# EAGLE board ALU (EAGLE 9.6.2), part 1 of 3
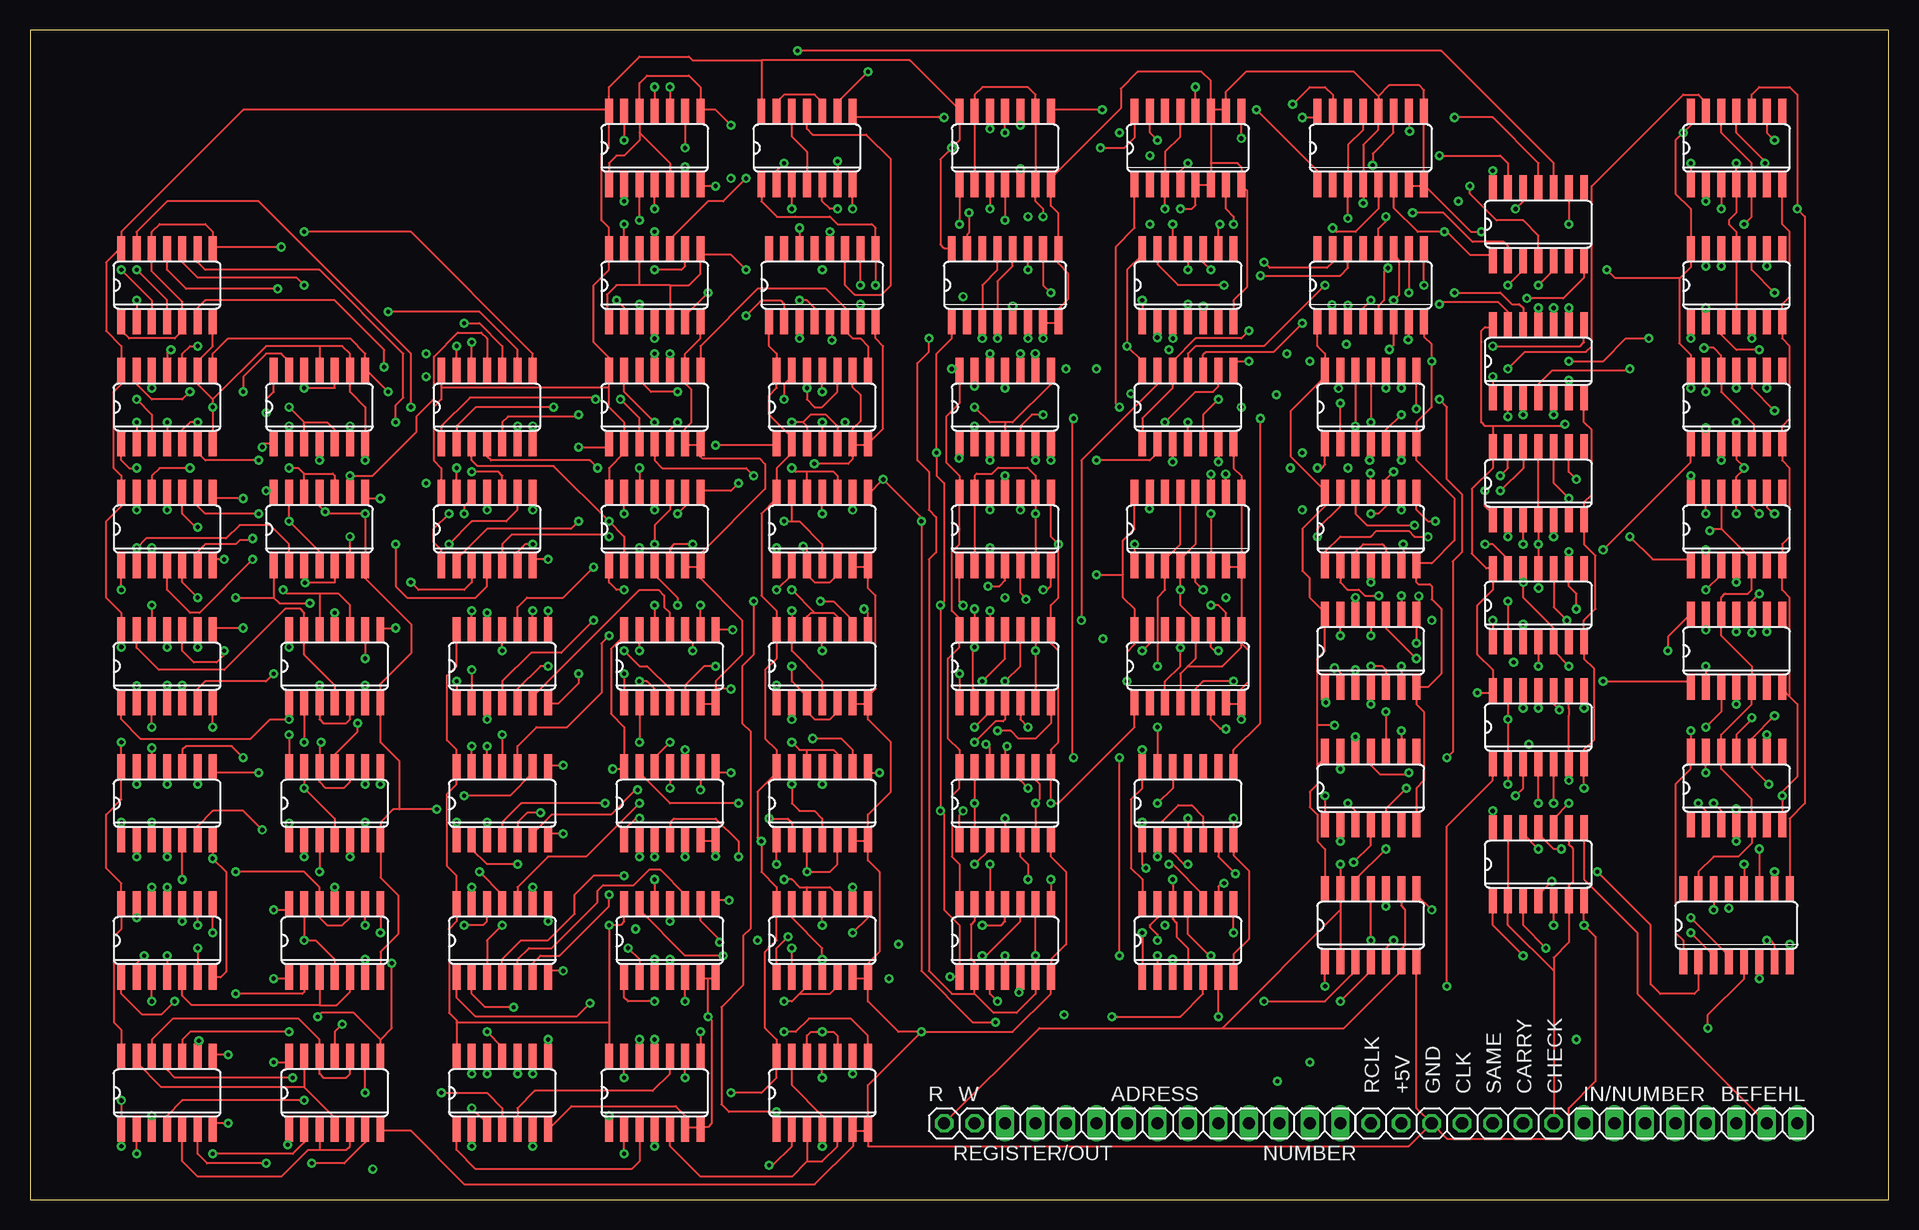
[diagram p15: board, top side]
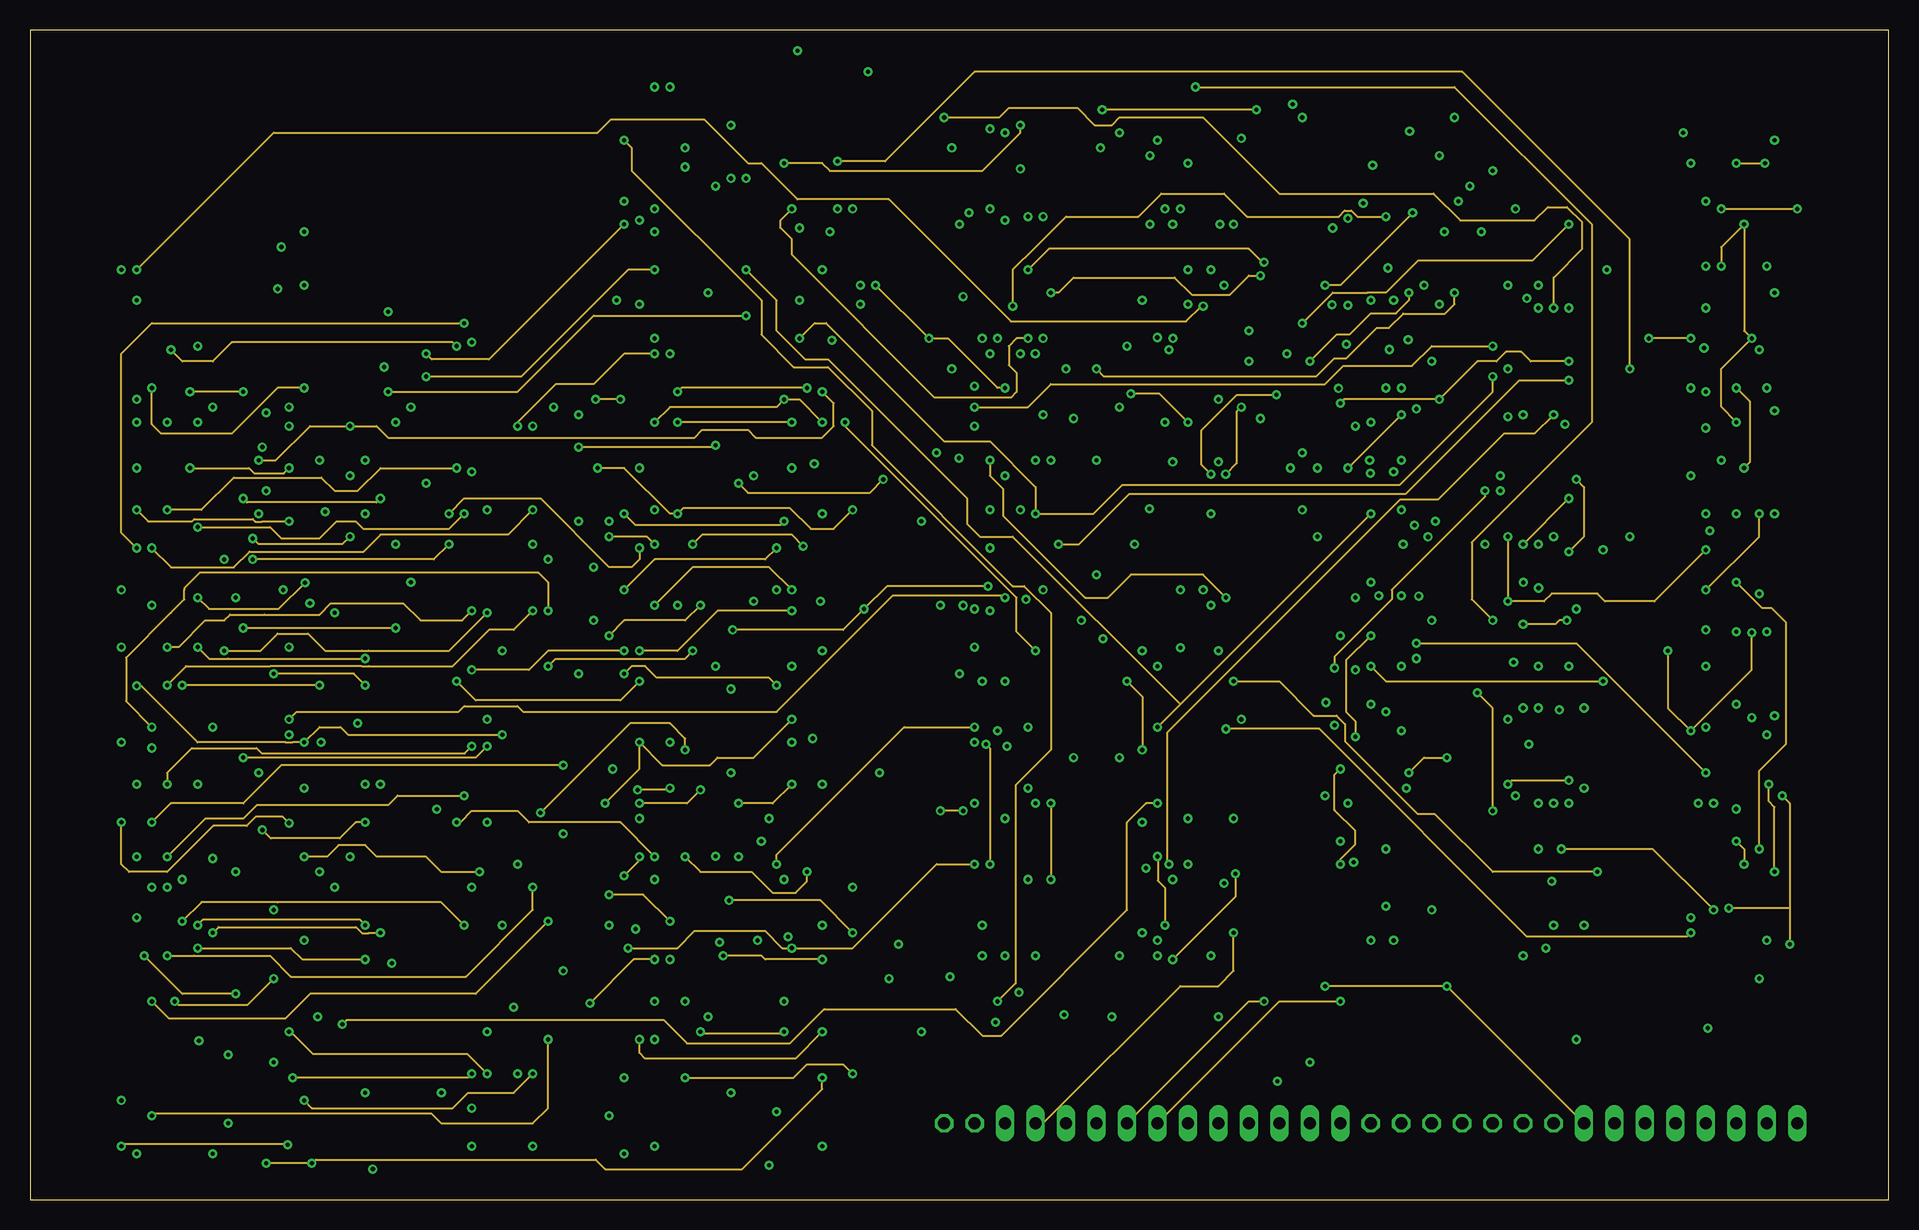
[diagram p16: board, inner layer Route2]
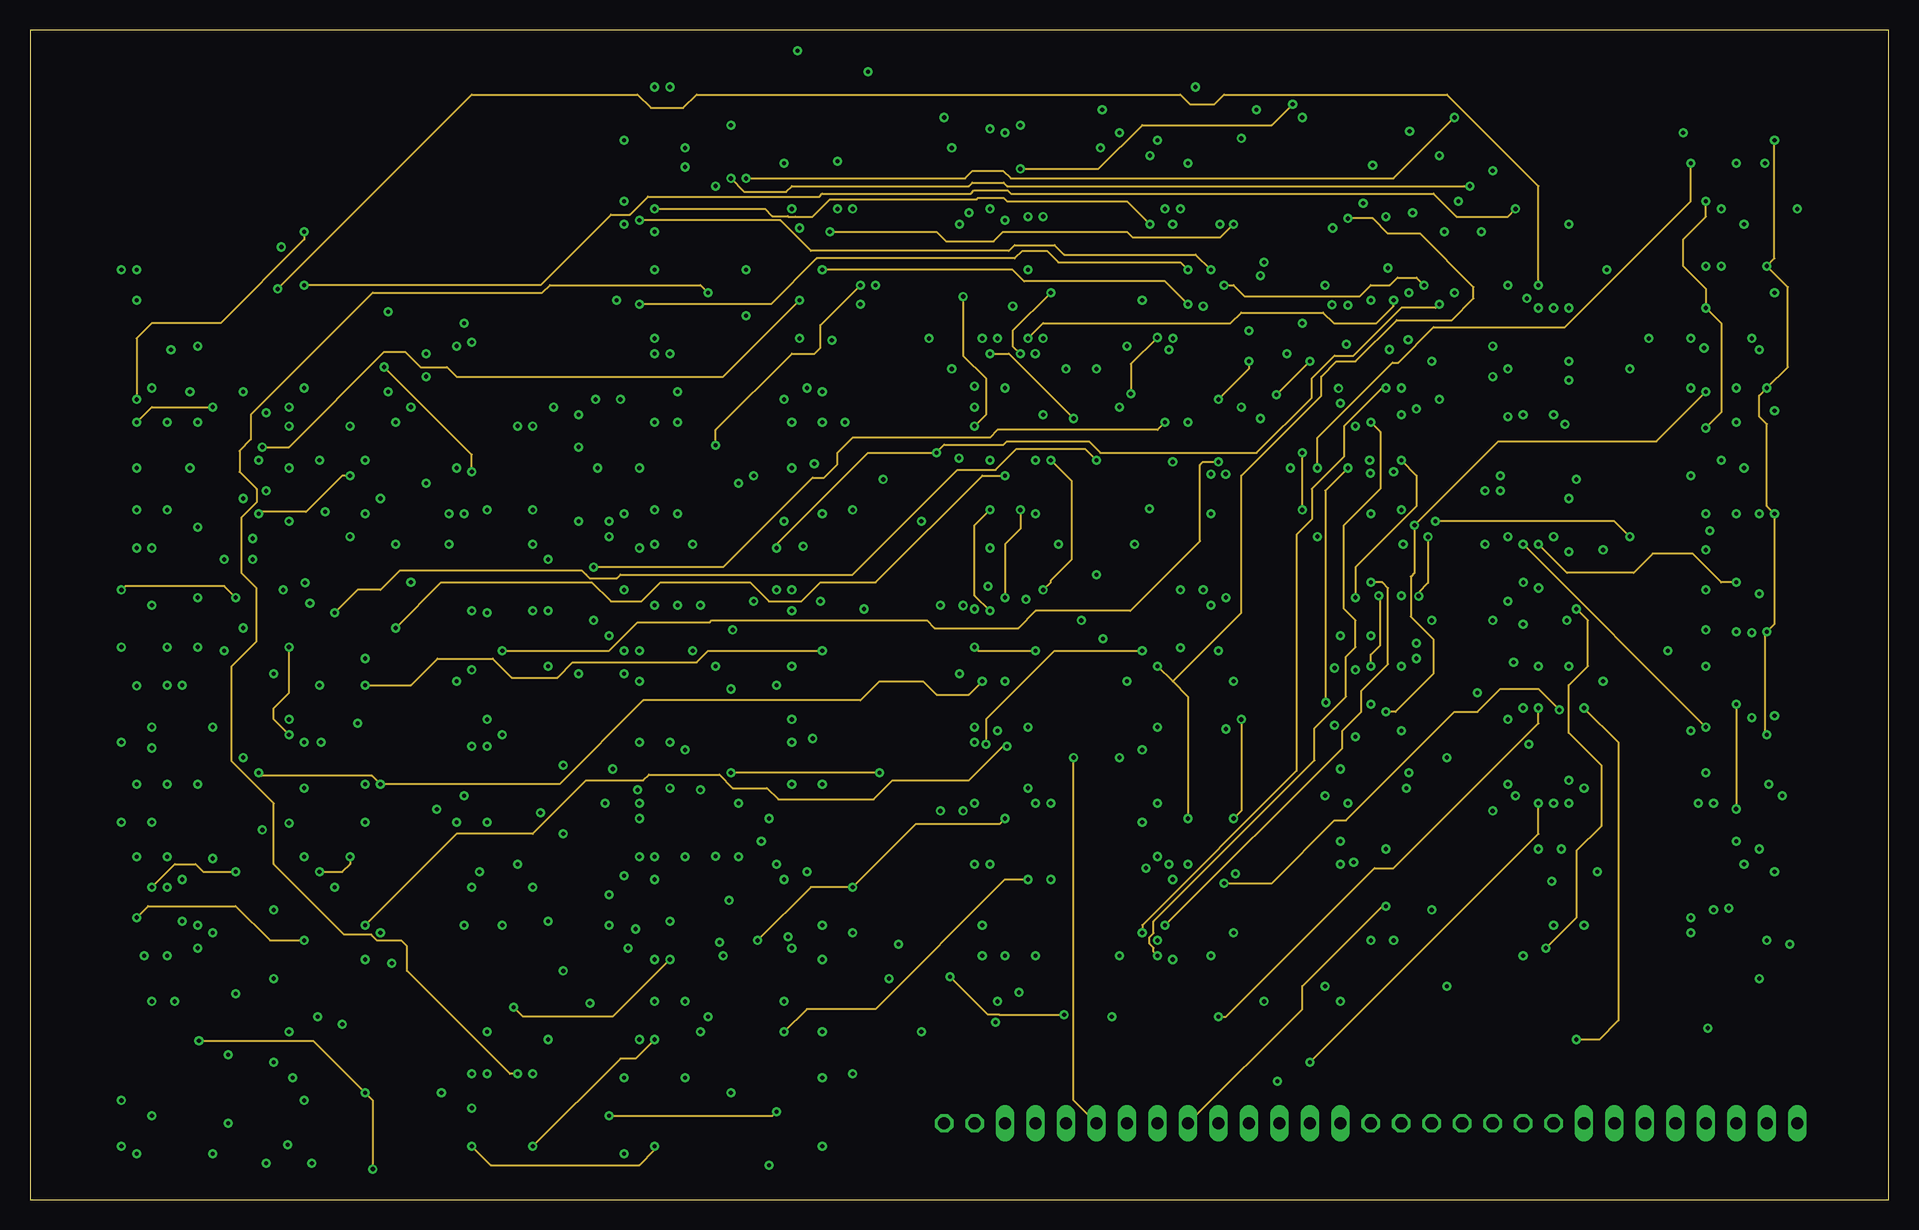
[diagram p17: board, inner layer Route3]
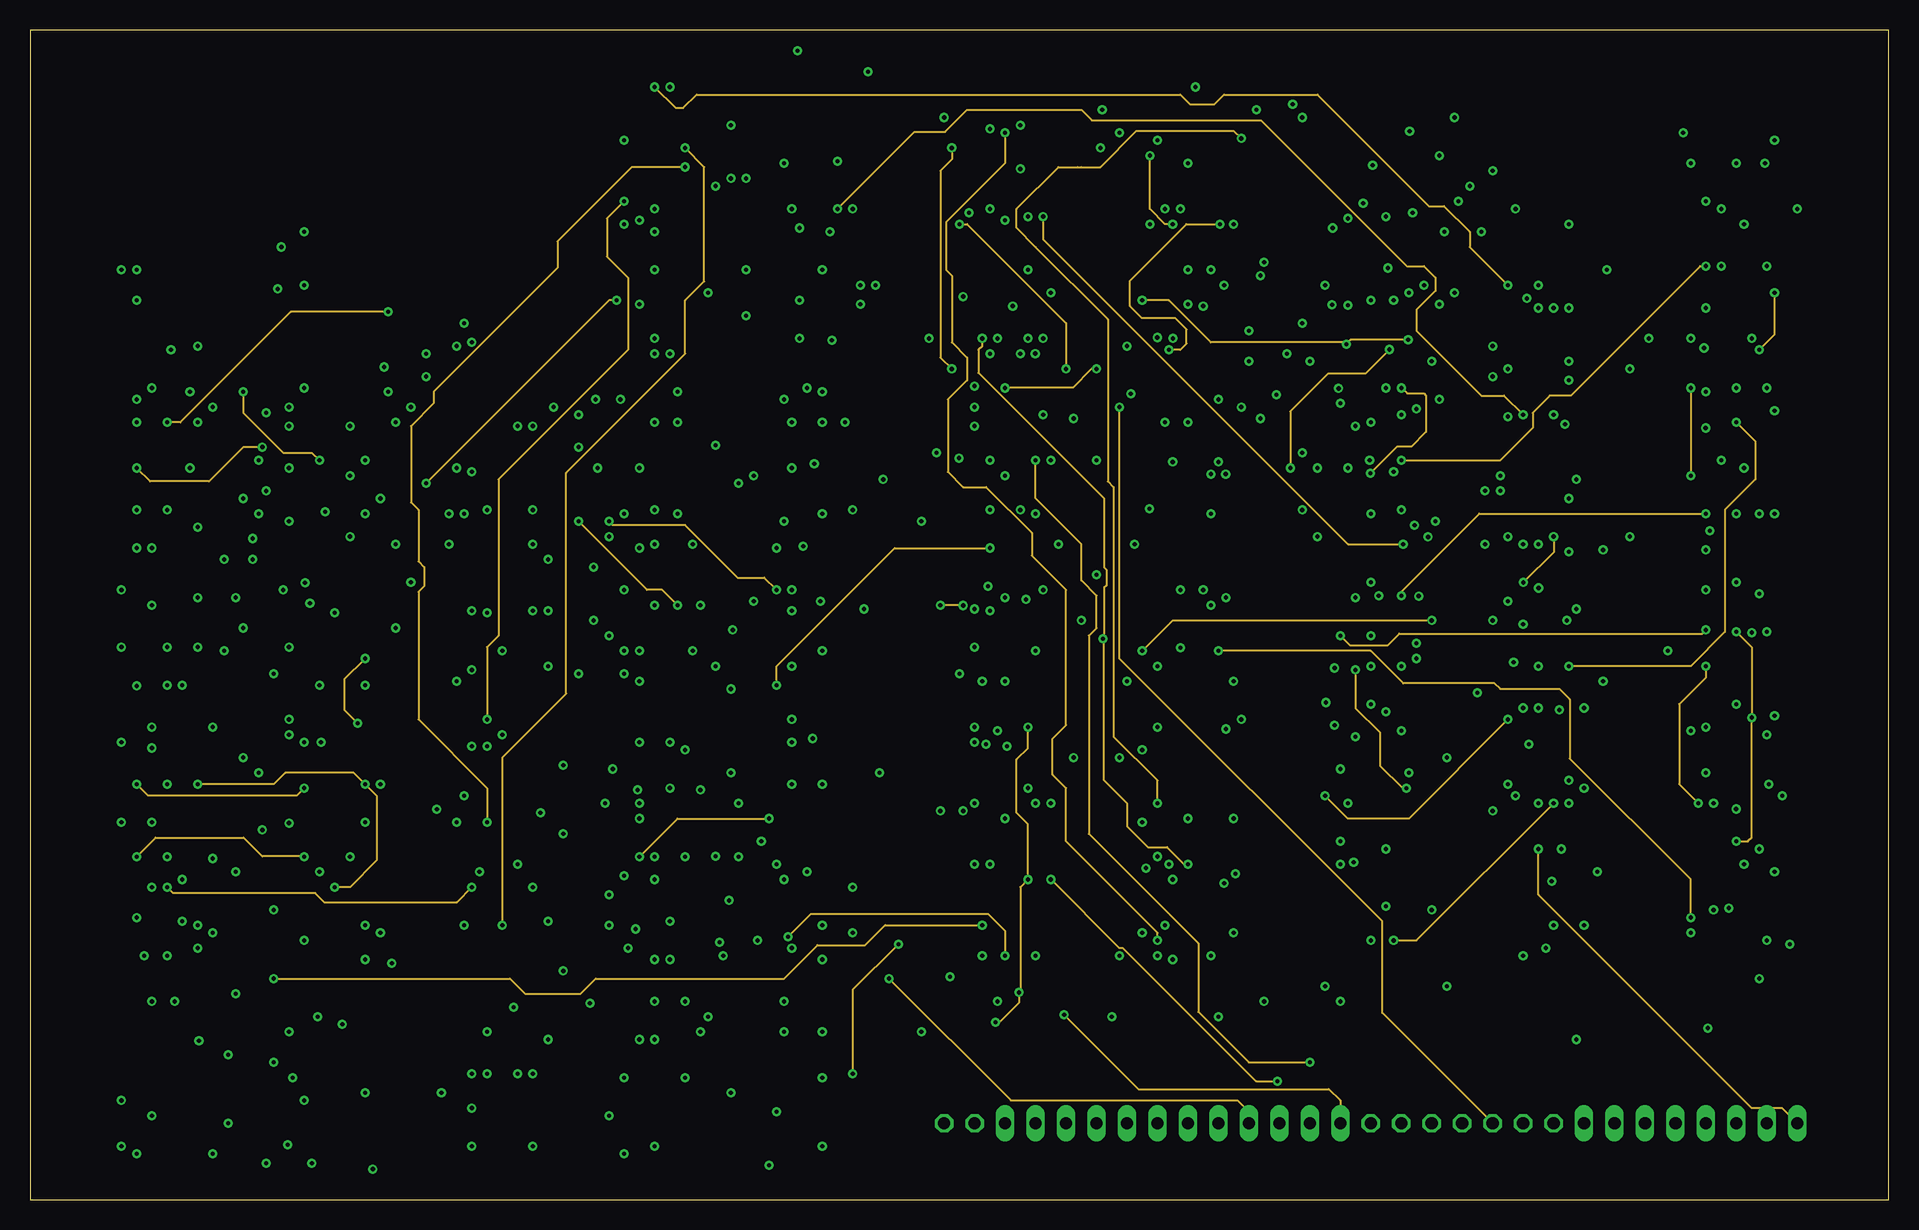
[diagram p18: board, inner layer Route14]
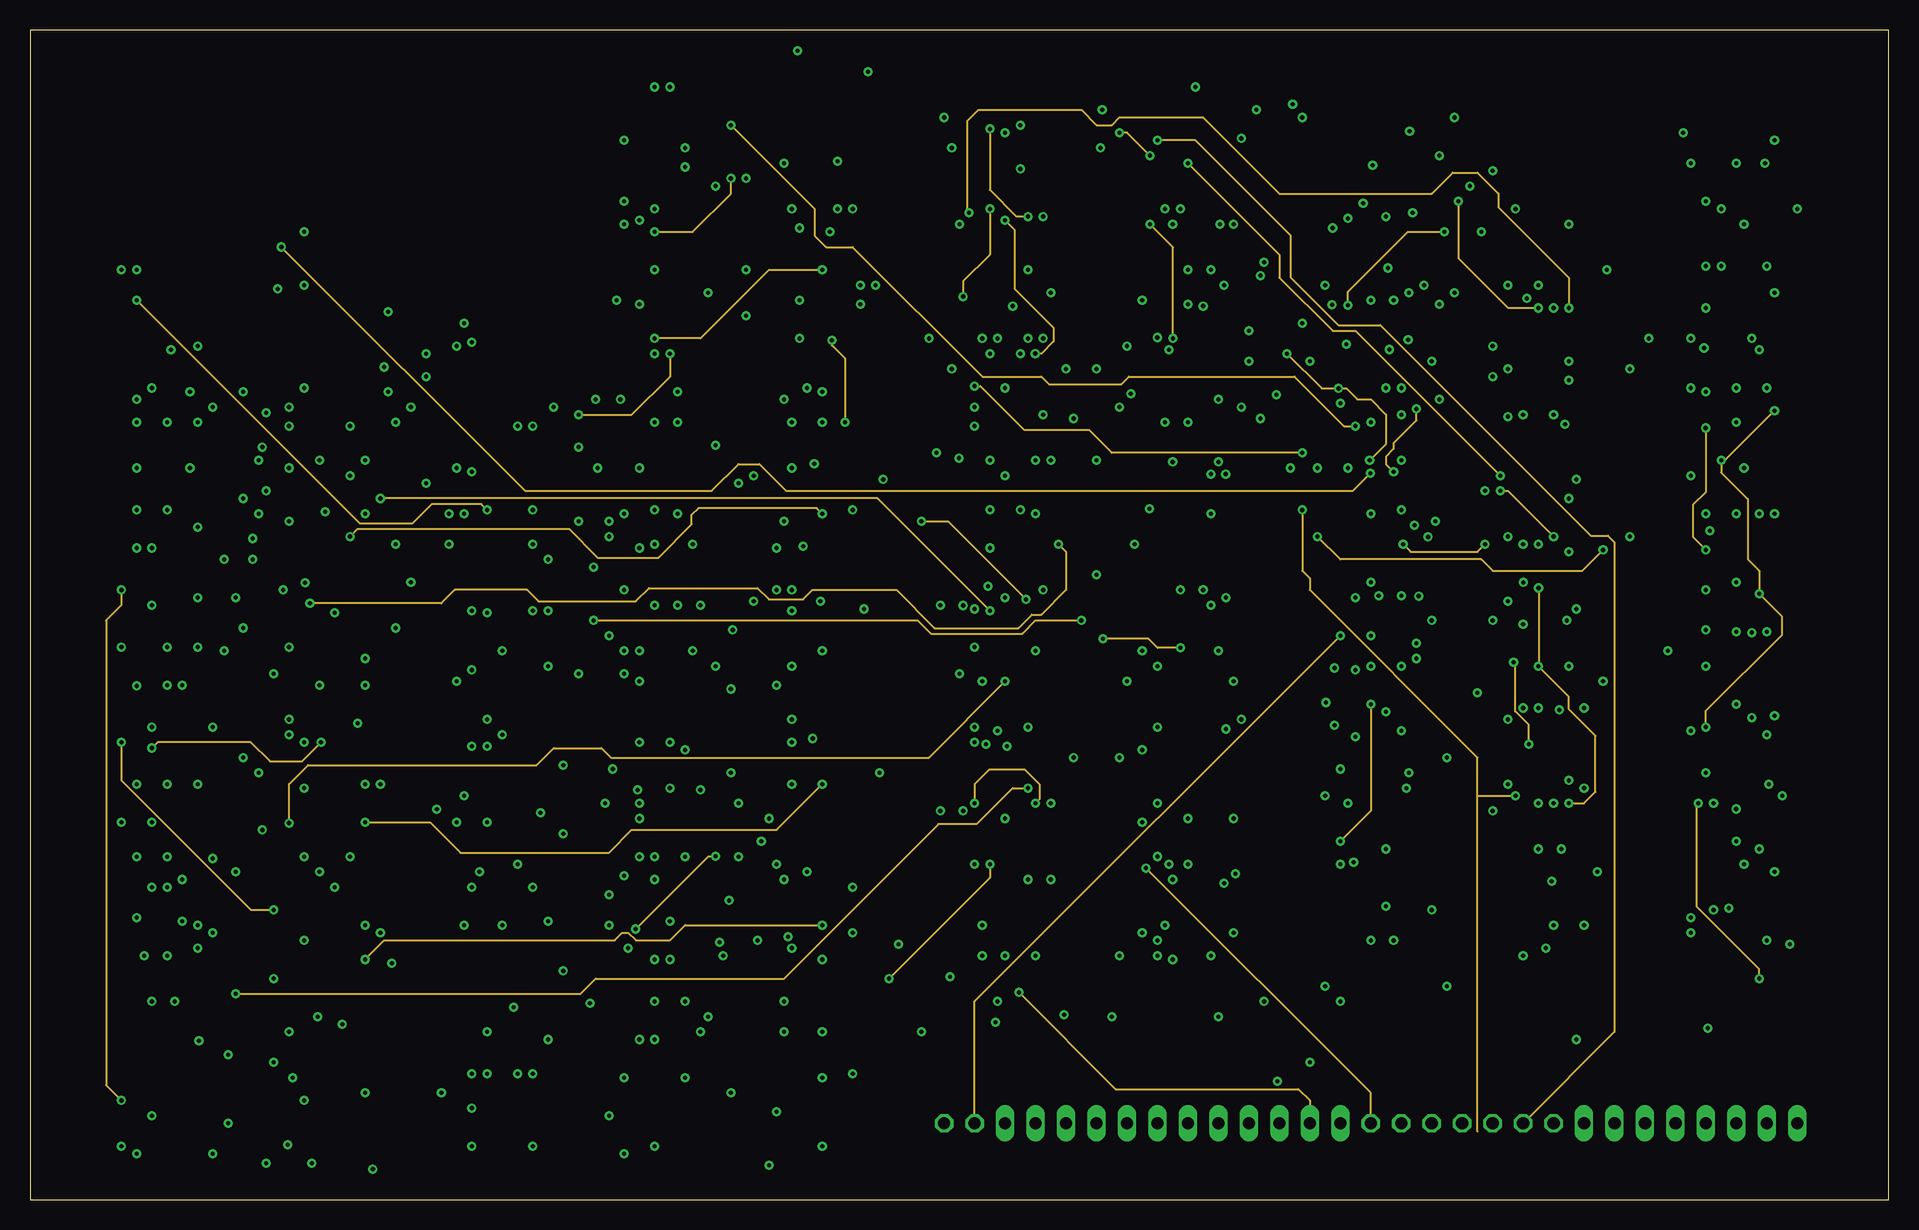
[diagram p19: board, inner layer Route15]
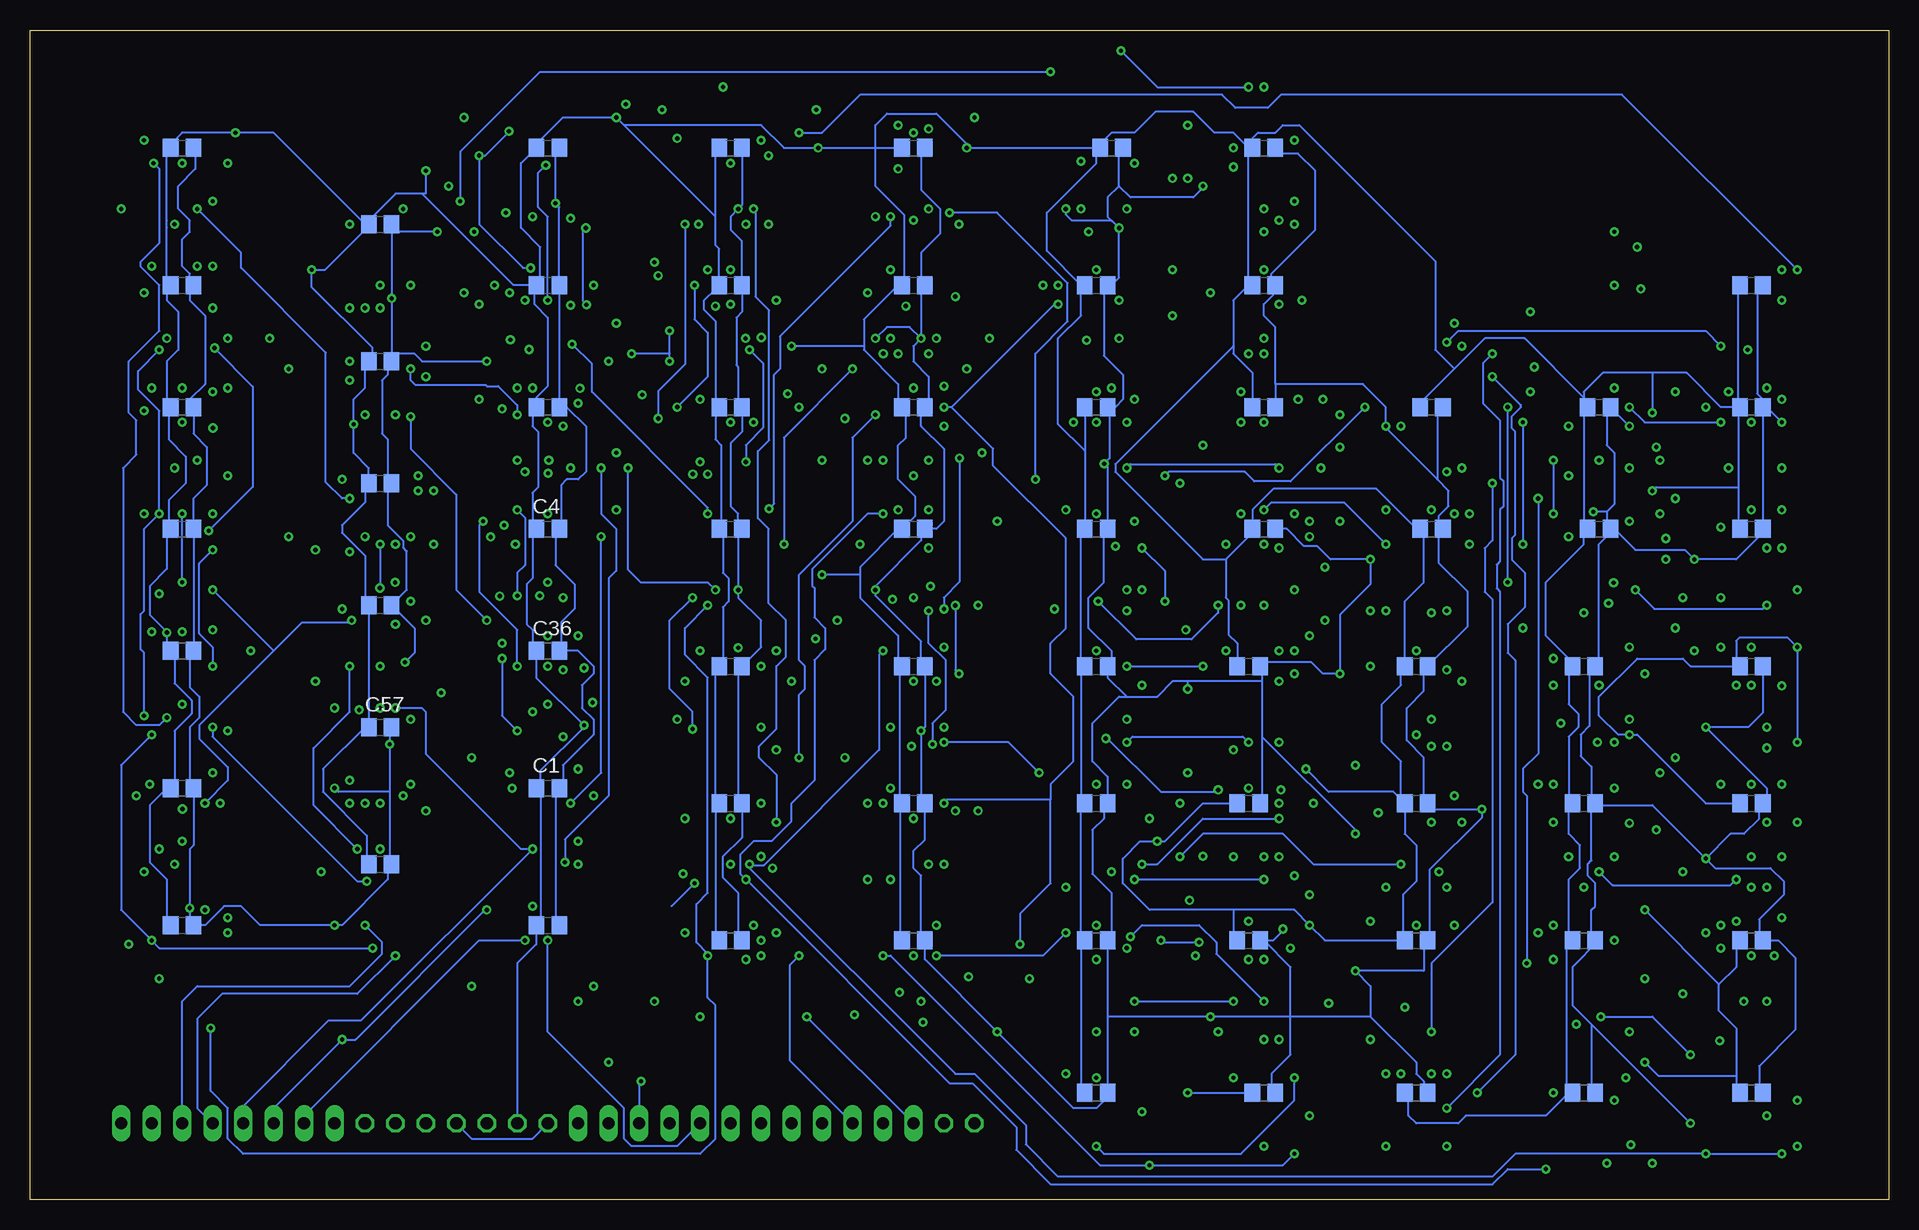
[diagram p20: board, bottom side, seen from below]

Size 154.92 x 97.46 mm. Coordinates in mm from the lower left corner, seen from the top.
Outline: 0,0 154.92,0 154.92,97.46 0,97.46 0,0
Copper layers (1+2*3+14*15+16): Top 0.035mm / dielectric 0.25mm / Route2 0.035mm / dielectric 0.25mm / Route3 0.035mm / dielectric 0.25mm / Route14 0.035mm / dielectric 0.25mm / Route15 0.035mm / dielectric 0.25mm / Bottom 0.035mm
Design rules "default *": minimum track width 6mil, minimum drill 0.35mm, track to track 8mil, track to pad 8mil, pad to pad 8mil, via to via 8mil, smd to smd 8mil, copper to edge 40mil, drill to drill 8mil, minimum pad ring 10mil, minimum via ring 8mil, stop-mask expansion 4mil, vias tented up to drill 0mil, thermal gap 10mil

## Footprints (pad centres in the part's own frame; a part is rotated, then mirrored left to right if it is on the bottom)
1X01 = drill 1.016 octagon: 1 0,0
1X04 = drill 1.016 long: 1 -3.81,0; 2 -1.27,0; 3 1.27,0; 4 3.81,0
C0805 = smd 1.3 x 1.5: 1 -0.95,0; 2 0.95,0
SO16 = smd 0.66 x 2.032: 1 -4.445,-3.073; 2 -3.175,-3.073; 3 -1.905,-3.073; 4 -0.635,-3.073; 5 0.635,-3.073; 6 1.905,-3.073; 7 3.175,-3.073; 8 4.445,-3.073; 9 4.445,3.073; 10 3.175,3.073; 11 1.905,3.073; 12 0.635,3.073; 13 -0.635,3.073; 14 -1.905,3.073; 15 -3.175,3.073; 16 -4.445,3.073
SO14 = smd 0.66 x 2.032: 1 -3.81,-3.073; 2 -2.54,-3.073; 3 -1.27,-3.073; 4 0,-3.073; 5 1.27,-3.073; 6 2.54,-3.073; 7 3.81,-3.073; 8 3.81,3.073; 9 2.54,3.073; 10 1.27,3.073; 11 0,3.073; 12 -1.27,3.073; 13 -2.54,3.073; 14 -3.81,3.073

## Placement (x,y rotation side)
+5V  [1X01]  114.3,6.35 0 top
ADRESS  [1X04]  95.25,6.35 0 top
BEFEHL  [1X04]  143.51,6.35 0 top
C1  [C0805]  111.76,34.29 0 bottom
C2  [C0805]  81.28,33.02 0 bottom
C3  [C0805]  96.52,33.02 0 bottom
C4  [C0805]  111.76,55.88 0 bottom
C5  [C0805]  142.24,76.2 0 bottom
C6  [C0805]  125.73,69.85 0 bottom
C7  [C0805]  111.76,76.2 0 bottom
C8  [C0805]  24.13,55.88 0 bottom
C9  [C0805]  38.1,55.88 0 bottom
C10  [C0805]  96.52,66.04 0 bottom
C11  [C0805]  111.76,22.86 0 bottom
C12  [C0805]  81.28,66.04 0 bottom
C13  [C0805]  66.04,66.04 0 bottom
C14  [C0805]  52.07,66.04 0 bottom
C15  [C0805]  96.52,76.2 0 bottom
C16  [C0805]  81.28,76.2 0 bottom
C17  [C0805]  52.07,76.2 0 bottom
C18  [C0805]  66.04,76.2 0 bottom
C19  [C0805]  52.07,87.63 0 bottom
C20  [C0805]  64.77,87.63 0 bottom
C21  [C0805]  81.28,87.63 0 bottom
C22  [C0805]  96.52,87.63 0 bottom
C23  [C0805]  11.43,76.2 0 bottom
C24  [C0805]  11.43,66.04 0 bottom
C26  [C0805]  39.37,44.45 0 bottom
C27  [C0805]  53.34,44.45 0 bottom
C29  [C0805]  24.13,66.04 0 bottom
C30  [C0805]  38.1,66.04 0 bottom
C31  [C0805]  11.43,55.88 0 bottom
C32  [C0805]  25.4,33.02 0 bottom
C33  [C0805]  11.43,33.02 0 bottom
C34  [C0805]  142.24,22.86 0 bottom
C35  [C0805]  142.24,34.29 0 bottom
C36  [C0805]  111.76,45.72 0 bottom
C37  [C0805]  142.24,45.72 0 bottom
C38  [C0805]  142.24,55.88 0 bottom
C39  [C0805]  96.52,55.88 0 bottom
C40  [C0805]  142.24,66.04 0 bottom
C41  [C0805]  125.73,81.28 0 bottom
C42  [C0805]  111.76,87.63 0 bottom
C43  [C0805]  66.04,55.88 0 bottom
C44  [C0805]  11.43,44.45 0 bottom
C45  [C0805]  25.4,44.45 0 bottom
C46  [C0805]  66.04,44.45 0 bottom
C47  [C0805]  66.04,21.59 0 bottom
C48  [C0805]  66.04,33.02 0 bottom
C49  [C0805]  53.34,33.02 0 bottom
C50  [C0805]  53.34,21.59 0 bottom
C51  [C0805]  39.37,21.59 0 bottom
C52  [C0805]  25.4,21.59 0 bottom
C53  [C0805]  39.37,33.02 0 bottom
C54  [C0805]  96.52,21.59 0 bottom
C55  [C0805]  81.28,21.59 0 bottom
C56  [C0805]  125.73,27.94 0 bottom
C57  [C0805]  125.73,39.37 0 bottom
C58  [C0805]  125.73,49.53 0 bottom
C59  [C0805]  125.73,59.69 0 bottom
C60  [C0805]  111.76,66.04 0 bottom
C61  [C0805]  142.24,87.63 0 bottom
C62  [C0805]  52.07,55.88 0 bottom
C63  [C0805]  81.28,55.88 0 bottom
C65  [C0805]  81.28,44.45 0 bottom
C66  [C0805]  96.52,44.45 0 bottom
C67  [C0805]  11.43,8.89 0 bottom
C68  [C0805]  25.4,8.89 0 bottom
C69  [C0805]  39.37,8.89 0 bottom
C70  [C0805]  52.07,8.89 0 bottom
C71  [C0805]  66.04,8.89 0 bottom
C72  [C0805]  11.43,21.59 0 bottom
CARRY  [1X01]  124.46,6.35 0 top
CHECK  [1X01]  127,6.35 0 top
CLK  [1X01]  119.38,6.35 0 top
GND  [1X01]  116.84,6.35 0 top
IC1  4027D  [SO16]  81.28,76.2 0 top
IC2  4049D  [SO16]  111.76,76.2 0 top
IC3  4027D  [SO16]  96.52,44.45 0 top
IC4  4049D  [SO16]  142.24,22.86 0 top
IC5  4027D  [SO16]  96.52,55.88 0 top
IC6  4081D  [SO14]  81.28,87.63 0 top
IC7  4027D  [SO16]  111.76,87.63 0 top
IC8  4071D  [SO14]  81.28,66.04 0 top
IC9  4071D  [SO14]  64.77,87.63 0 top
IC10  4081D  [SO14]  96.52,33.02 0 top
IC11  4070D  [SO14]  66.04,8.89 0 top
IC12  4081D  [SO14]  52.07,8.89 0 top
IC13  4071D  [SO14]  39.37,8.89 0 top
IC14  4070D  [SO14]  25.4,8.89 0 top
IC15  4081D  [SO14]  11.43,8.89 0 top
IC16  4081D  [SO14]  52.07,55.88 0 top
IC17  4070D  [SO14]  66.04,55.88 0 top
IC18  4071D  [SO14]  38.1,55.88 0 top
IC19  4070D  [SO14]  24.13,55.88 0 top
IC20  4081D  [SO14]  11.43,55.88 0 top
IC21  4081D  [SO14]  52.07,66.04 0 top
IC22  4070D  [SO14]  66.04,66.04 0 top
IC23  4071D  [SO14]  38.1,66.04 0 top
IC24  4070D  [SO14]  24.13,66.04 0 top
IC25  4081D  [SO14]  11.43,66.04 0 top
IC26  4049D  [SO16]  66.04,76.2 0 top
IC27  4081D  [SO14]  81.28,21.59 0 top
IC28  4081D  [SO14]  81.28,33.02 0 top
IC29  4081D  [SO14]  81.28,44.45 0 top
IC30  4081D  [SO14]  81.28,55.88 0 top
IC31  4081D  [SO14]  53.34,21.59 0 top
IC32  4070D  [SO14]  66.04,21.59 0 top
IC33  4071D  [SO14]  39.37,21.59 0 top
IC34  4070D  [SO14]  25.4,21.59 0 top
IC35  4081D  [SO14]  11.43,21.59 0 top
IC36  4081D  [SO14]  53.34,33.02 0 top
IC37  4070D  [SO14]  66.04,33.02 0 top
IC38  4071D  [SO14]  39.37,33.02 0 top
IC39  4070D  [SO14]  25.4,33.02 0 top
IC40  4081D  [SO14]  11.43,33.02 0 top
IC41  4081D  [SO14]  53.34,44.45 0 top
IC42  4070D  [SO14]  66.04,44.45 0 top
IC43  4071D  [SO14]  39.37,44.45 0 top
IC44  4070D  [SO14]  25.4,44.45 0 top
IC45  4081D  [SO14]  11.43,44.45 0 top
IC47  4027D  [SO16]  96.52,87.63 0 top
IC48  4081D  [SO14]  11.43,76.2 0 top
IC49  4081D  [SO14]  52.07,76.2 0 top
IC50  4081D  [SO14]  52.07,87.63 0 top
IC51  4081D  [SO14]  96.52,66.04 0 top
IC52  4070D  [SO14]  125.73,69.85 0 top
IC53  4072D  [SO14]  125.73,81.28 0 top
IC54  4072D  [SO14]  96.52,76.2 0 top
IC55  4082D  [SO14]  142.24,34.29 0 top
IC56  4082D  [SO14]  142.24,45.72 0 top
IC57  4082D  [SO14]  142.24,55.88 0 top
IC58  4082D  [SO14]  142.24,66.04 0 top
IC59  4082D  [SO14]  142.24,76.2 0 top
IC60  4082D  [SO14]  142.24,87.63 0 top
IC61  4082D  [SO14]  125.73,49.53 0 top
IC62  4082D  [SO14]  125.73,59.69 0 top
IC63  4081D  [SO14]  125.73,39.37 0 top
IC64  4081D  [SO14]  125.73,27.94 0 top
IC65  4081D  [SO14]  111.76,22.86 0 top
IC66  4072D  [SO14]  111.76,34.29 0 top
IC67  4071D  [SO14]  111.76,45.72 0 top
IC68  4071D  [SO14]  111.76,55.88 0 top
IC69  4071D  [SO14]  111.76,66.04 0 top
IC70  4071D  [SO14]  96.52,21.59 0 top
IN/NUMBER  [1X04]  133.35,6.35 0 top
NUMBER  [1X04]  105.41,6.35 180 top
R  [1X01]  76.2,6.35 0 top
RCLK  [1X01]  111.76,6.35 0 top
REGISTER/OUT  [1X04]  85.09,6.35 180 top
SAME  [1X01]  121.92,6.35 0 top
W  [1X01]  78.74,6.35 0 top

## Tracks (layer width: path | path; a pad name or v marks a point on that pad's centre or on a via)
1AKKU/N0  (via drill 0.35)
  Top 0.152: v63.5,82.55 IC9.3 | IC1.6 v83.19,71.75 | v113.67,74.93 114.14,75.41 114.14,78.26 113.67,78.74 IC2.11
  Route2 0.152: v63.5,82.55 62.55,81.6 62.55,80.96 63.5,80.01 63.5,78.74 75.41,66.83 81.76,66.83 82.23,67.31 82.23,68.9 81.6,69.53 81.6,71.12 82.23,71.75 v83.19,71.75
  Route3 0.152: v83.19,71.75 84.45,73.03 100.08,73.03 100.97,73.91 107.79,73.91 108.68,73.03 112.24,73.03 113.67,74.45 v113.67,74.93
1AKKU/N1  (via drill 0.35)
  Top 0.152: IC1.10 84.45,76.2 v85.09,75.56 | v102.55,76.99 109.22,76.99 109.86,77.63 IC2.14 | IC8.10 v82.55,70.48
  Route2 0.152: v85.09,75.56 85.72,75.56 87,76.84 95.41,76.84 96.84,75.41 100.01,75.41 101.6,76.99 v102.55,76.99
  Route3 0.152: v82.55,70.48 81.92,71.12 81.92,72.39 v85.09,75.56
1AKKU/N2  (via drill 0.35)
  Top 0.152: IC3.6 98.42,40.01 99.22,39.21 v99.69,39.21 | v138.43,22.22 140.34,20.32 IC4.3 | v80.01,61.59 IC8.3
  Route2 0.152: v99.69,39.21 107.47,39.21 124.78,21.91 138.11,21.91 v138.43,22.22 | v80.01,61.59 80.01,60.33 81.12,59.21 81.12,56.99 87.95,50.16 89.85,50.16 91.76,52.07 97.79,52.07 v99.69,50.16
  Bottom 0.152: v99.69,39.21 99.69,40.64 101.6,42.55 101.6,48.26 v99.69,50.16
1AKKU/N3  (via drill 0.35)
  Top 0.152: v98.42,20.32 98.32,20.32 96.52,22.12 IC70.11 | v98.42,49.53 99.06,49.53 99.69,48.9 IC3.10 | v139.86,14.29 139.86,15.4 142.88,18.41 IC4.5
  Bottom 0.152: v139.86,14.29 139.86,9.05 138.43,7.62 138.43,5.08 137.16,3.81 99.06,3.81 97.79,5.08 97.79,16.19 98.42,16.83 v98.42,20.32 98.42,20.48 99.38,21.43 99.38,24.61 98.42,25.56 98.42,43.5 100.33,45.4 100.33,47.62 v98.42,49.53
1AKKU/WRITE  (via drill 0.35)
  Top 0.152: IC68.4 v111.76,51.44 | IC10.2 v93.98,28.59 v93.97,28.58
  Route2 0.152: v93.97,28.58 94.01,28.55 94.01,26.58 94.61,25.97 v94.61,22.86
  Route3 0.152: v94.61,22.86 109.38,37.62 109.38,39.05 110.97,40.64 110.97,42.39 113.19,44.61 113.19,50.96 112.71,51.44 v111.76,51.44
2AKKU/O0  (via drill 0.35)
  Top 0.152: IC9.2 62.23,85.73 v62.87,86.36 | IC6.10 v82.55,89.53
  Route2 0.152: v62.87,86.36 66.04,86.36 66.67,85.73 79.38,85.73 82.55,88.9 v82.55,89.53
2AKKU/O1  (via drill 0.35)
  Top 0.152: IC6.4 v81.28,81.6 | v83.79,70.5 83.82,70.47 IC8.9
  Route15 0.152: v81.28,81.6 82.07,80.8 82.07,75.88 85.33,72.63 85.33,71.52 84.3,70.48 83.81,70.48 v83.79,70.5
2AKKU/O2  (via drill 0.35)
  Top 0.152: v78.74,64.45 IC8.2 | IC6.3 v80.01,82.55
  Route3 0.152: v78.74,64.45 79.69,65.41 79.69,68.42 77.79,70.33 v77.79,75.25
  Route15 0.152: v80.01,82.55 80.01,78.74 77.79,76.52 v77.79,75.25
2AKKU/O3  (via drill 0.35)
  Top 0.152: v81.28,88.9 IC6.11 | IC70.13 93.98,23.49 93.34,22.86 93.34,22.7 93.98,22.07 v93.98,21.59
  Route14 0.152: v81.28,88.9 81.28,86.36 76.36,81.44 76.36,77.47 76.83,76.99 76.83,71.44 78.11,70.17 78.11,68.26 76.52,66.67 76.52,60.64 77.79,59.37 79.69,59.37 83.5,55.56 83.5,53.66 86.36,50.8 86.36,39.53 85.25,38.42 85.25,35.4 86.36,34.29 86.36,29.84 93.98,22.22 v93.98,21.59
2AKKU/WRITE  (via drill 0.35)
  Top 0.152: v100.49,27.15 99.06,28.57 IC10.6 | v95.25,20 IC70.3
  Route2 0.152: v100.49,27.15 100.49,25.24 v95.25,20
+5V  (via drill 0.35)
  Top 0.152: IC27.14 77.47,27.94 76.83,28.57 76.83,33.66 77.47,34.29 IC28.14 77.47,37.47 76.52,38.42 76.52,45.09 77.47,46.04 IC29.14 77.47,48.42 76.83,49.05 76.83,53.98 77.47,54.61 IC30.14 77.47,60.33 76.36,61.44 76.36,65.25 77.47,66.36 IC8.14 77.47,69.22 v76.83,69.22 | 60.96,94.93 IC9.14 | 60.96,94.93 73.34,94.93 77.47,90.81 IC6.14 77.47,88.27 v76.83,87.63 75.88,86.68 75.88,79.59 76.2,79.27 IC1.16 | v20.32,11.43 21.59,11.43 IC14.14 | v20.32,24.13 21.59,24.13 IC34.14 | v21.59,38.73 IC39.14 | IC15.14 7.62,14.13 6.99,14.76 6.99,21.91 7.62,22.54 IC35.14 7.62,26.35 6.35,27.62 6.35,32.07 7.62,33.34 IC40.14 v7.62,38.1 | IC18.14 34.29,60.96 33.66,61.59 33.66,66.04 34.29,66.67 34.29,67.63 | IC23.14 34.29,67.63 | IC16.14 48.26,60.96 49.53,62.23 IC21.2 49.53,64.77 48.26,66.04 48.26,67.63 | 48.26,67.63 IC21.14 48.26,70.17 46.99,71.44 46.99,76.2 48.26,77.47 IC49.14 48.26,80.96 47.62,81.6 47.62,87 48.26,87.63 IC50.14 | IC50.14 48.26,90.81 17.78,90.81 7.62,80.64 IC48.14 7.52,79.27 6.35,78.11 6.35,72.39 7.62,71.12 IC25.14 7.62,67.95 6.99,67.31 6.99,60.96 7.62,60.33 IC20.14 7.62,57.79 6.35,56.52 6.35,50.16 7.62,48.9 IC45.14 v7.62,46.04 | 48.26,67.63 34.29,67.63 | 60.96,94.93 55.24,94.93 54.93,95.25 50.8,95.25 48.26,92.71 IC50.14 | v19.68,65.56 19.68,66.67 20.32,67.31 IC24.14 | v58.42,8.89 60.96,8.89 62.23,10.16 IC11.14 62.23,13.34 61.28,14.29 61.28,20.64 62.23,21.59 IC32.14 62.23,26.04 60.96,27.3 v60.96,29.84 60.64,30.16 60.64,33.97 62.23,35.56 IC37.14 62.23,37.47 61.28,38.42 61.28,44.13 62.23,45.09 IC42.14 62.23,49.05 60.96,50.32 60.96,57.15 62.23,58.42 IC17.14 62.23,60.96 63.5,62.23 IC22.2 63.5,63.5 61.59,65.41 61.59,66.99 62.23,67.63 IC22.14 62.23,70.48 61.59,71.12 IC26.1
  Top 0.152: 48.26,14.76 v48.26,22.86 49.21,22.86 49.53,23.18 IC31.14 | 48.26,14.76 IC12.14 | IC41.14 49.53,46.99 48.42,45.88 48.42,40.48 49.53,39.37 IC36.14 49.53,35.88 v48.58,35.88 | 35.56,14.76 35.56,14.92 34.92,15.56 34.92,22.54 35.56,23.18 IC33.14 35.56,26.99 34.77,27.78 34.77,33.81 35.56,34.61 IC38.14 35.56,37.47 34.77,38.26 34.77,43.66 35.56,44.45 IC43.14 | 35.56,14.76 IC13.14 | 35.56,14.76 48.26,14.76 | IC4.1 137.79,21.59 137.16,22.22 137.16,34.61 138.43,35.88 IC55.14 v138.43,39.05 | IC60.14 138.43,89.53 v137.79,88.9 137.16,88.27 137.16,83.82 138.43,82.55 IC59.14 138.43,77.69 137.53,76.78 | IC57.14 v138.43,60.33 | 137.53,76.78 137.48,76.73 137.48,71.34 138.43,70.38 IC58.14 v138.43,67.63 | IC70.14 92.71,26.67 91.76,27.62 91.76,33.34 92.71,34.29 IC10.14 v92.71,37.47 | v91.44,43.18 91.44,45.62 92.08,46.25 IC3.16 92.08,49.21 91.12,50.16 91.12,52.07 | IC5.16 92.08,55.88 91.12,54.93 91.12,52.07 | IC51.14 92.71,69.85 v91.44,71.12 91.44,77.47 92.71,78.74 IC54.14 | v88.9,52.07 91.12,52.07 | v106.05,90.17 107.31,90.17 IC7.16 | v121.92,85.73 IC53.14 | IC2.1 107.31,71.12 107.95,70.48 IC69.14 107.95,68.58 105.09,65.72 105.09,61.91 107.95,59.05 IC68.14 107.95,57.79 106.05,55.88 106.05,52.39 106.68,51.75 106.68,50.16 107.95,48.9 IC67.14 107.95,45.72 107.31,45.09 107.31,39.53 | IC65.14 107.95,29.21 107.31,29.84 107.31,32.07 106.68,32.7 106.68,33.97 107.31,34.61 107.31,36.2 | 107.31,36.2 107.95,36.83 IC66.14 | 107.31,36.2 107.31,39.53 | v108.74,39.53 107.31,39.53 | v19.69,59.05 20.23,59.05 IC19.14 | IC44.14 v21.59,46.04 | v89.22,87.63 91.22,87.63 92.08,88.48 IC47.16 | 137.53,76.78 132.13,76.78 v131.44,77.47
  Top 0.152: IC64.14 v121.92,32.38 | v120.65,42.23 121.92,42.23 IC63.14 121.92,44.13 120.65,45.4 120.65,49.53 121.92,50.8 IC61.14 121.39,52.6 120.17,53.82 120.17,59.21 121.92,60.96 IC62.14 121.92,64.45 | IC56.14 136.53,46.89 v136.53,45.72 | v127.95,64.61 127.79,64.45 121.92,64.45 | 121.92,64.45 121.28,64.45 120.97,64.77 120.97,72.39 121.28,72.71 121.7,72.71 IC52.14
  Route2 0.152: v91.44,43.18 92.71,41.91 v92.71,37.47 | v121.92,32.38 121.92,40.96 v120.65,42.23 | v136.53,45.72 136.53,40.96 v138.43,39.05 143.51,44.13 v143.51,47.25
  Route3 0.152: v21.59,46.04 21.59,42.23 20.32,40.96 20.32,40.01 v21.59,38.73
  Route14 0.152: v76.83,87.63 76.83,86.68 75.88,85.73 75.88,70.17 v76.83,69.22 | v138.43,67.63 v138.43,60.33
  Route15 0.152: v20.32,24.13 18.41,24.13 7.62,34.92 v7.62,38.1
  Bottom 0.152: 12.7,10.32 12.7,14.29 14.13,15.72 14.13,17.94 | 12.7,10.32 12.7,8.89 C67.1 | C72.1 12.7,21.59 12.7,19.37 14.13,17.94 | v20.32,11.43 19.21,10.32 12.7,10.32 | v20.32,24.13 14.13,17.94 | C33.1 15.24,33.02 20.95,38.73 v21.59,38.73 22.54,38.73 24.13,40.32 24.13,41.91 20.95,45.09 17.14,45.09 16.51,44.45 12.7,44.45 | C44.1 12.7,44.45 | v7.62,38.1 v7.62,46.04 8.38,46.8 12.45,46.8 12.7,46.55 12.7,44.45 | 25.4,66.04 25.4,55.88 | 36.2,69.22 38.73,66.67 38.73,66.04 C30.1 | 25.4,66.04 C29.1 | 12.54,65.72 12.54,59.37 | 12.54,59.37 12.54,55.88 C31.1 | 12.54,66.04 12.54,76.2 C23.1 | 12.54,66.04 12.7,66.04 12.7,65.41 12.54,65.72 | 12.54,66.04 C24.1 | 12.54,65.72 C24.1 | 25.4,66.83 25.4,67.31 23.81,68.9 19.68,68.9 | 25.4,66.83 25.4,66.04 | 26.67,33.02 26.67,38.58 25.88,39.37 25.88,40.48 26.67,41.28 26.67,44.45 C45.1 26.04,44.45 28.57,46.99 28.57,51.44 25.4,54.61 25.4,55.88 | 26.67,8.89 26.67,9.05 26.83,9.21 26.83,21.59 26.67,21.59 | 26.67,8.89 28.57,6.98 35.24,6.98 35.88,6.35 39.37,6.35 40.01,6.98 40.01,8.89 C69.1 | 26.67,8.89 C68.1 | 26.67,21.59 26.67,26.67 25.72,27.62 25.72,29.53 26.67,30.48 26.67,33.02 | 26.67,33.02 C32.1 | 26.67,21.59 C52.1 | 25.4,55.88 C8.1 | v58.42,8.89 C70.1 | C49.1 57.15,33.02 60.33,29.84 v60.96,29.84 62.39,29.84 63.82,28.42 63.82,26.35 61.59,24.13 54.61,24.13 | C53.1 40.64,33.02 40.64,36.51 42.23,38.1 42.23,41.28 40.64,42.86 40.64,44.45 C26.1 40.32,49.85 38.73,51.44 38.73,55.88 C9.1 39.37,55.88 42.7,59.21 51.28,59.21 53.02,57.47 53.02,55.56 | 55.24,53.34 55.24,50.16 55.01,49.93 55.01,47.07 54.29,46.36 C27.1 | 53.02,55.56 52.7,55.88 C62.1 | 53.02,55.56 55.24,53.34
  Bottom 0.152: 54.61,71.12 54.61,74.93 53.34,76.2 | 54.61,71.12 54.61,70.48 53.02,68.9 C14.1 | 53.34,76.2 53.34,87.63 | 53.34,76.2 C17.1 | 53.34,87.63 54.61,88.9 56.2,88.9 57.94,90.65 61.12,90.65 62.87,88.9 64.77,88.9 65.41,88.27 65.41,87.63 C20.1 66.04,87.63 | 53.34,87.63 C19.1 53.02,88.43 52.55,88.9 51.12,88.9 50.48,89.53 49.12,89.53 37.78,78.2 37.78,70.8 36.2,69.22 | 66.99,62.39 C43.1 | 67.31,76.2 67.31,73.66 69.22,71.75 69.22,64.61 66.99,62.39 | C13.1 66.99,62.39 | 67.31,44.45 67.31,33.02 | 67.31,21.59 67.31,8.89 C71.1 | 67.31,21.59 67.31,33.02 | 67.31,33.02 C48.1 | 67.31,21.59 C47.1 | 67.31,44.45 67.31,55.88 C43.1 | C43.1 | 67.31,44.45 C46.1 | 66.04,87.63 66.04,86.36 70.17,82.23 70.17,79.06 67.31,76.2 | 67.31,76.2 C18.1 | 55.24,53.34 57.15,53.34 64.45,60.64 64.45,61.28 54.61,71.12 | 82.39,33.02 82.39,21.59 C55.1 | 82.39,33.02 82.39,44.45 | 82.39,33.02 C2.1 | 85.41,71.12 85.41,73.34 82.55,76.2 82.39,76.2 | 85.41,71.12 85.41,70.8 82.55,67.95 82.55,66.04 C12.1 81.92,66.04 81.92,63.5 82.55,62.87 82.55,60.01 81.12,58.58 81.12,56.99 C63.1 82.55,55.88 85.72,52.71 85.72,52.07 | 82.39,76.2 C16.1 | 85.72,52.07 85.72,50.16 82.55,46.99 82.55,44.45 82.39,44.45 | 82.39,44.45 C65.1 | 85.41,71.12 v91.44,71.12 | 85.72,52.07 v88.9,52.07 | 97.79,33.02 97.79,21.59 C54.1 | 97.79,33.02 97.79,44.45 C66.1 97.16,44.45 97.16,49.37 96.68,49.85 96.68,51.75 97.16,52.23 97.16,55.88 C39.1 97.31,56.04 97.31,62.87 97.79,63.34 97.79,66.04 | 97.79,33.02 C3.1 | 97.79,66.04 C10.1 | 97.79,81.92 97.79,79.53 97.47,79.21 C15.1 97.79,76.2 97.79,75.86 98.77,74.89 98.77,74.18 97.79,73.21 97.79,66.04 | 97.79,81.92 97.79,87.63 C22.1 | 97.79,81.92 105.41,89.53
  Bottom 0.152: 105.41,89.53 v106.05,90.17 110.49,90.17 113.03,87.63 C42.1 113.98,86.36 113.98,80.96 112.39,79.38 112.39,76.2 | C34.1 143.51,22.86 143.51,26.67 144.94,28.1 144.94,32.86 143.51,34.29 C35.1 142.88,34.29 142.88,39.05 141.45,40.48 141.45,41.59 142.88,43.02 142.88,45.72 C37.1 143.51,45.72 v143.51,47.25 143.51,47.31 144.94,48.74 144.94,51.12 143.51,52.55 143.51,55.88 143.35,55.88 | 143.51,76.2 143.51,74.93 142.56,73.98 142.56,70.8 143.51,69.85 143.51,66.04 143.35,66.04 | 143.51,76.2 C5.1 | 143.35,55.88 143.35,58.26 141.92,59.69 141.92,61.91 143.35,63.34 143.35,66.04 | 143.35,55.88 C38.1 | 143.35,66.04 C40.1 | C56.1 126.84,27.94 126.84,30.32 130.49,33.97 130.49,35.88 127,39.37 C57.1 | 127,81.28 124.46,83.82 122.24,83.82 | v121.92,85.73 121.92,83.82 122.24,83.82 | C58.1 C57.1 | C57.1 | C58.1 127,49.53 127,53.66 128.91,55.56 128.91,56.2 127,58.1 127,59.69 C59.1 126.68,60.96 127.95,62.23 v127.95,64.61 127.95,66.67 127,67.63 127,69.85 C6.1 126.36,69.85 126.36,70.96 131.44,76.04 v131.44,77.47 130.33,77.47 126.68,81.12 C41.1 127,81.28 | C58.1 | +5V.1 114.3,19.68 112.71,21.27 C11.1 112.37,22.86 112.37,34.29 112.39,34.29 | 113.03,55.88 113.03,51.75 113.51,51.28 113.51,47.94 113.03,47.47 113.03,45.72 C36.1 112.71,43.5 v108.74,39.53 108.74,39.37 112.39,35.72 112.39,34.29 | 113.03,55.88 113.03,58.9 112.55,59.37 112.55,63.98 113.03,64.45 113.03,66.04 C60.1 112.71,66.84 111.76,67.79 111.76,73.5 112.87,74.61 112.87,75.72 112.39,76.2 | 113.03,55.88 C4.1 | 112.39,34.29 C1.1 | 122.24,83.82 114.62,76.2 C7.1 112.39,76.2 | 127,81.28 134.62,88.9 v137.79,88.9 142.24,88.9 142.88,88.27 142.88,87.63 C61.1 143.51,87.63 143.51,81.58 143.53,81.55 143.53,81.01 143.51,80.98 143.51,76.2
  Bottom 0.152: 84.45,87.63 v89.22,87.63 92.08,87.63 93.98,89.53 105.41,89.53 | 84.45,87.63 C21.1 | 66.04,87.63 v76.83,87.63 76.83,87.95 79.38,90.49 83.5,90.49 84.45,89.53 84.45,87.63 | 12.54,59.37 19.37,59.37 v19.69,59.05 | 84.45,87.63 84.45,84.45 82.07,82.07 82.07,76.52 82.39,76.2 | C24.1 13.97,66.04 16.83,68.9 19.68,68.9 | C53.1 41.27,33.97 46.67,33.97 v48.58,35.88 | 40.48,21.59 46.99,21.59 v48.26,22.86 49.53,24.13 54.61,24.13 | 40.48,21.59 C51.1 | 54.61,24.13 54.61,21.91 C50.1 | 19.68,68.9 v19.68,65.56 | 25.4,66.83 30.32,71.75 33.66,71.75 36.2,69.22 | C53.1 40.32,30.48 39.37,29.53 39.37,26.51 40.48,25.4 40.48,21.59
A/IN/N0  (via drill 0.35)
  Top 0.152: IC65.3 110.49,19.05 107.95,16.51 v102.87,16.51
  Route2 0.152: v102.87,16.51 101.6,16.51 ADRESS.1
A/IN/N1  (via drill 0.35)
  Top 0.152: IC65.4 111.76,19.05 v109.22,16.51
  Route2 0.152: v109.22,16.51 104.14,16.51 ADRESS.2
A/IN/N2  (via drill 0.35)
  Top 0.152: v113.03,24.45 IC65.10
  Route3 0.152: ADRESS.3 106.05,15.88 106.05,17.78 112.71,24.45 v113.03,24.45
A/IN/N3  (via drill 0.35)
  Top 0.152: v111.76,21.59 IC65.11
  Bottom 0.152: v111.76,21.59 111.76,13.97 105.41,7.62 105.41,5.08 104.78,4.45 100.97,4.45 ADRESS.4
ADA  (via drill 0.35)
  Top 0.152: v114.3,50.32 IC67.9 | v114.3,57.47 IC68.9 | v139.7,57.15 IC57.13
  Route14 0.152: v139.7,57.15 120.81,57.15 114.3,50.64 v114.3,50.32
  Bottom 0.152: v114.3,57.47 113.67,56.83 113.67,52.86 114.3,52.23 v114.3,50.32
ADD/OUT/CARRY  (via drill 0.35)
  Top 0.152: IC14.11 25.4,13.97 v26.04,14.61 | v93.98,33.02 95.25,34.29 IC10.12 | v100.97,88.42 IC47.9
  Route2 0.152: v93.98,33.02 93.03,33.02 91.44,31.43 91.44,24.13 80.96,13.65 79.38,13.65 77.15,15.88 66.2,15.88 63.34,13.02 54.77,13.02 52.84,14.95 26.38,14.95 v26.04,14.61
  Route14 0.152: v93.98,33.02 93.98,34.92 90.33,38.58 90.33,59.37 89.85,59.85 89.85,73.34 83.82,79.38 82.23,80.96 82.23,82.55 85.72,86.04 87.31,86.04 87.63,86.04 89.22,86.04 92.23,89.06 100.33,89.06 v100.97,88.42
ADD/OUT/N0  (via drill 0.35)
  Top 0.152: v36.83,7.62 38.1,6.35 IC13.3 | IC49.13 v49.53,81.28
  Route2 0.152: v33.02,70.48 33.5,70.01 38.26,70.01 v49.53,81.28
  Bottom 0.152: v36.83,7.62 32.38,12.07 32.38,50.64 32.66,50.92 32.66,52.9 32.38,53.18 32.38,57.47 32.11,57.75 32.11,59.89 32.38,60.17 32.38,64.93 33.81,66.36 33.81,69.69 v33.02,70.48
ADD/OUT/N1  (via drill 0.35)
  Top 0.152: v34.29,8.89 38.1,8.89 39.37,7.62 IC13.4 | v52.07,77.47 54.29,77.47 54.61,77.79 IC49.9
  Route2 0.152: v33.02,68.58 40.96,68.58 49.85,77.47 v52.07,77.47
  Bottom 0.152: v34.29,8.89 31.11,12.07 31.11,44.93 31.75,45.56 31.75,47.94 30.32,49.37 30.32,52.23 31.39,53.3 31.39,55.12 31.11,55.4 31.11,63.98 31.39,64.26 31.39,65.28 30.64,66.04 30.64,66.2 v33.02,68.58
ADD/OUT/N2  (via drill 0.35)
  Top 0.152: v56.52,75.56 54.61,73.66 IC49.6 | v40.64,10.48 IC13.10
  Route3 0.152: v40.64,10.48 40.01,10.48 31.43,19.05 31.43,21.11 30.98,21.57 28.94,21.57 28.44,22.07 26.19,22.07 20.32,27.94 20.32,33.02 16.83,36.51 16.83,44.45 18.89,46.51 18.89,50.96 17.62,52.23 17.62,56.83 18.89,58.1 18.89,59.21 17.46,60.64 17.46,62.39 18.41,63.34 18.41,65.41 28.57,75.56 42.7,75.56 43.34,76.2 55.88,76.2 v56.52,75.56
ADD/OUT/N3  (via drill 0.35)
  Top 0.152: IC13.11 39.37,12.7 v38.1,13.97 | v48.9,74.93 49.53,74.3 IC49.2
  Route14 0.152: v33.02,59.69 48.26,74.93 v48.9,74.93
  Bottom 0.152: v38.1,13.97 38.1,19.68 33.02,24.76 33.02,50.01 33.66,50.64 33.66,54.29 33.02,54.93 v33.02,59.69
ADN  (via drill 0.35)
  Top 0.152: v114.3,44.45 IC67.6 | v117.16,56.52 116.52,56.52 115.57,57.47 IC68.8 | v133.35,55.25 135.25,53.34 138.43,53.34 IC57.1
  Route3 0.152: v133.35,55.25 132.08,56.52 v117.16,56.52
  Bottom 0.152: v114.3,44.45 114.3,47.47 117.47,50.64 117.47,56.2 v117.16,56.52
ALU/IN/Z1/N0  (via drill 0.35)
  Top 0.152: IC30.1 77.47,49.85 77.79,49.53 v77.79,49.5 | IC12.1 v48.26,6.98 | IC16.1 48.26,51.44 48.9,50.8 v49.53,50.8 | v62.23,54.29 IC17.1 | IC52.13 123.19,73.98 122.4,74.77 117.63,74.77 v117.47,74.61 | IC1.1 76.83,71.75 75.56,70.48 v75.56,62.23 75.56,60.33 76.2,59.69 76.2,49.85 v75.88,49.53 v75.88,32.38 76.2,32.07 76.2,24.13 77.47,22.86 IC27.1 77.41,18.57 v76.68,18.57 | IC11.1 v62.23,7.3 58.26,7.3 57.63,7.94 57.63,16.03 59.45,17.86 59.45,21.99 60.09,22.62 60.09,38.97 59.37,39.69 59.37,44.45 60.33,45.4 v60.33,49.85 | v77.47,43.82 IC29.1 | IC28.1 77.47,32.01 77.79,32.33 v77.79,32.38
  Route2 0.152: v49.53,50.8 52.07,53.34 61.28,53.34 v62.23,54.29 | v77.79,32.38 v75.88,32.38
  Route3 0.152: v117.47,74.61 117.16,74.3 114.3,74.3 110.33,70.33 108.74,70.33 106.84,68.42 106.84,66.83 102.23,62.23 89.22,62.23 88.27,63.18 81.44,63.18 81.16,62.9 76.2,62.9 75.56,62.27 v75.56,62.23 69.85,62.23 62.23,54.61 v62.23,54.29 | v48.26,6.98 61.91,6.98 v62.23,7.3 | v86.2,15.4 80.78,15.4 80.76,15.42 79.83,15.42 v76.68,18.57
  Route14 0.152: v77.79,49.5 75.91,49.5 v75.88,49.53 | v86.2,15.4 92.39,9.21 108.27,9.21 109.22,8.26 NUMBER.1
  Bottom 0.152: v60.33,49.85 60.33,52.39 v62.23,54.29 | v77.79,49.5 77.79,44.13 v77.47,43.82
ALU/IN/Z1/N1  (via drill 0.35)
  Top 0.152: v55.88,13.97 IC12.8 | v62.87,13.97 63.82,13.97 64.93,15.08 68.42,15.08 69.85,13.65 IC11.8 | v83.19,26.67 83.19,27.94 82.55,28.57 IC28.5 | v59.05,59.69 58.42,59.05 55.88,59.05 IC16.8 | IC17.8 69.85,58.74 v71.12,60.01 74.3,56.83 v74.3,56.52 74.3,19.05 78.58,14.76 v80.49,14.76 | v78.26,82.23 78.26,80.54 78.11,80.39 IC1.15 | IC30.5 82.55,50.58 83.03,50.11 v83.03,50.01 | v128.27,74.3 IC52.9 | IC29.5 82.55,40.01 v83.19,39.37 | v82.44,17.26 82.44,18.41 IC27.5
  Route2 0.152: v55.88,13.97 56.04,13.81 62.71,13.81 v62.87,13.97 | v59.05,59.69 59.85,58.9 70.01,58.9 v71.12,60.01
  Route3 0.152: v62.87,13.97 64.77,15.88 70.48,15.88 81.28,26.67 v83.19,26.67
  Route14 0.152: v83.19,39.37 83.19,37.62 82.23,36.67 82.23,32.23 83.19,31.27 v83.19,26.67 82.55,26.04 82.55,17.37 v82.44,17.26 82.44,16.4 80.8,14.76 v80.49,14.76
  Route15 0.152: v83.03,50.01 76.52,56.52 v74.3,56.52 | v128.27,74.3 128.27,76.84 122.4,82.71 122.4,83.82 120.65,85.57 118.59,85.57 116.84,83.82 104.14,83.82 97.79,90.17 90.81,90.17 90.17,89.53 88.9,89.53 87.63,90.81 79.06,90.81 78.11,89.85 78.11,82.39 v78.26,82.23 | v82.44,17.26 90.49,9.21 105.73,9.21 106.68,8.26 NUMBER.2
  Bottom 0.152: v71.12,60.01 71.12,70.48 68.42,73.18 68.42,76.36 74.3,82.23 v78.26,82.23
ALU/IN/Z1/N2  (via drill 0.35)
  Top 0.152: v7.62,4.45 IC15.1 v7.62,8.26 | v7.62,50.8 IC20.1 | IC19.1 20.32,50.16 | v85.09,26.67 IC27.8 | IC3.1 92.08,39.37 85.72,33.02 v85.09,33.02 IC28.8 85.09,37.47 85.72,38.1 85.72,45.72 85.09,46.36 IC29.8 85.09,49.53 85.72,50.16 v85.72,54.61 85.09,55.25 IC30.8 | v128.27,68.26 IC52.6 | v23.34,49.69 20.8,49.69 20.32,50.16 | v17.14,50.16 20.32,50.16 | v21.48,4.56 21.48,5.71 IC14.1
  Route2 0.152: v128.27,68.26 124.14,68.26 114.68,58.8 91.63,58.8 87.44,54.61 v85.72,54.61 | v21.48,4.56 21.43,4.6 7.78,4.6 v7.62,4.45 | v85.09,33.02 v85.09,26.67
  Route3 0.152: v7.62,50.8 7.94,51.12 16.19,51.12 v17.14,50.16
  Route14 0.152: v85.09,26.67 90.78,20.98 91.08,20.98 102.19,9.87 v103.98,9.87
  Route15 0.152: v23.34,49.69 34.29,49.69 35.4,50.8 41.43,50.8 42.39,49.85 50.48,49.85 51.59,50.96 60.64,50.96 61.59,50.01 64.45,50.01 65.25,50.8 72.23,50.8 75.41,47.62 82.39,47.62 83.5,48.74 84.3,48.74 86.36,50.8 86.36,53.98 v85.72,54.61 | v7.62,50.8 7.62,49.53 6.35,48.26 6.35,9.53 v7.62,8.26
  Bottom 0.152: v103.98,9.87 104.14,9.71 NUMBER.3
ALU/IN/Z1/N3  (via drill 0.35)
  Top 0.152: v17.78,58.42 15.24,58.42 IC20.8 | v29.21,58.42 27.94,58.42 IC19.8 | v16.51,12.07 15.24,12.07 IC15.8 | v23.97,15.24 24.29,15.56 26.99,15.56 29.21,13.34 | IC14.8 29.21,13.34 | v30.16,19.68 30.16,14.29 29.21,13.34 | v80.01,49.05 IC29.12 | v80.01,27.94 IC27.12 | IC28.12 80.01,37.68 79.75,37.94 v79.69,37.94 | IC3.15 93.34,46.36 v92.71,45.72 | v123.19,65.25 IC52.2 | IC30.12 v80.01,57.48
  Route2 0.152: v29.21,58.42 28.89,58.1 18.1,58.1 v17.78,58.42 | v79.69,37.94 80.01,37.62 v80.01,27.94
  Route3 0.152: v80.01,49.05 78.74,50.32 78.74,56.21 v80.01,57.48 | v79.69,37.94 79.69,40.01 85.41,45.72 v92.71,45.72
  Route14 0.152: v116.84,48.26 95.25,48.26 v92.71,45.72 | v71.6,18.41 81.76,8.26 100.65,8.26 101.6,7.3 NUMBER.4
  Route15 0.152: v29.21,58.42 70.64,58.42 v80.01,49.05 | v80.01,27.94 80.01,26.83 v71.6,18.41
  Bottom 0.152: v23.97,15.24 19.68,15.24 v16.51,12.07 | v30.16,19.68 30.16,33.66 30.48,33.97 30.48,35.88 29.21,37.15 v29.21,58.42 | v123.19,65.25 123.19,62.55 119.38,58.74 119.38,50.8 v116.84,48.26 | v80.01,49.05 80.01,46.36 78.58,44.93 78.58,40.8 79.69,39.69 v79.69,37.94
ALU/IN/Z2/N0  (via drill 0.35)
  Top 0.152: IC27.13 78.74,23.23 78.42,22.92 78.42,20.1 78.74,19.79 IC27.2 78.74,17.14 | v49.53,3.81 IC12.2 | IC11.2 63.5,4.45 61.91,2.86 v61.59,2.86 | IC27.9 v83.82,20.32 IC27.6 83.82,17.14 82.23,15.56 80.33,15.56 78.74,17.14 | IC9.1 60.96,83.19 62.25,81.89 63.77,81.89 63.8,81.92 66.67,81.92 67.31,81.28 70.17,81.28 70.48,80.96 IC26.9 v70.48,76.2 | v81.28,67.63 IC8.11 | IC52.12 124.46,74.3 124.14,74.61 123.51,74.61 122.56,75.56 v118.75,75.56 | 78.74,17.14 76.83,17.14 74.93,19.05 74.93,53.34 75.53,53.94 75.53,56.87 74.93,57.47 74.93,60.64 73.98,61.59 73.98,69.69 74.93,70.64 v74.93,71.75
  Route2 0.152: v70.48,76.2 v74.93,71.75 76.52,71.75 80.64,67.63 v81.28,67.63 | v88.9,69.22 89.53,68.58 107.19,68.58 108.71,70.1 109.73,70.1 112.27,72.64 113.28,72.64 114.46,73.82 117.95,73.82 118.75,74.61 v118.75,75.56
  Route14 0.152: v88.9,69.22 88.49,69.22 86.93,67.66 81.31,67.66 v81.28,67.63
  Bottom 0.152: v49.53,3.81 50.48,2.86 v61.59,2.86 65.72,2.86 83.19,20.32 v83.82,20.32
ALU/IN/Z2/N1  (via drill 0.35)
  Top 0.152: IC28.2 v78.74,33.02 IC28.13 | v54.61,10.16 IC12.9 | v68.58,10.48 IC11.9 | IC8.8 85.09,67.95 81.92,64.77 81.28,64.77 | 81.28,64.77 IC8.4 | v69.22,74.61 IC26.7 | v121.92,71.12 129.22,71.12 129.54,71.44 IC52.8 | 81.28,64.77 80.01,64.77 v78.74,66.04 | IC28.9 83.82,34.98 84.14,34.66 84.14,33.34 v83.82,33.02 IC28.6
  Route2 0.152: v54.61,10.16 63.66,10.16 64.77,11.27 67.79,11.27 v68.58,10.48 | v121.92,71.12 116.84,71.12 115.19,69.47 109.47,69.47 107.95,67.95 85.09,67.95 83.19,66.04 v78.74,66.04
  Route14 0.152: v72.39,21.27 68.58,17.46 v68.58,10.48
  Route15 0.152: v83.82,33.02 84.14,33.34 84.14,34.61 82.9,35.85 79.98,35.85 78.74,34.61 v78.74,33.02
  Bottom 0.152: v69.22,74.61 69.53,74.61 78.11,66.04 | v78.74,33.02 78.42,33.34 69.85,33.34 | 69.85,33.34 69.85,34.61 67.94,36.51 67.94,41.91 69.85,43.82 69.85,46.36 68.58,47.62 68.58,55.09 74.64,61.15 74.64,62.58 78.11,66.04 | v72.39,21.27 72.39,23.81 69.85,26.35 69.85,33.34 | 78.11,66.04 v78.74,66.04
ALU/IN/Z2/N2  (via drill 0.35)
  Top 0.152: IC29.2 78.74,42.49 78.58,42.65 78.58,45.88 v78.74,46.04 IC29.13 v78.74,49.21 | IC29.9 v83.82,45.72 IC29.6 | v8.89,3.81 IC15.2 | v15.24,3.81 21.91,3.81 22.86,4.76 IC14.2 | IC70.10 97.79,25.4 95.25,27.94 v94.93,27.94 | v127,65.41 IC52.5 | IC26.5 66.84,72.96 v66.84,71.6 | IC8.1 77.47,61.82 v77.44,61.79
  Route2 0.152: v67.94,64.77 67.94,64.45 82.23,50.16 82.23,47.31 v83.82,45.72 | v127,65.41 125.41,63.82 122.87,63.82 117.4,58.34 114.22,58.34 94.77,38.89 94.77,27.94 v94.93,27.94
  Route3 0.152: v78.74,46.04 79.06,45.72 v83.82,45.72
  Route15 0.152: v66.84,71.6 66.84,71.18 67.92,70.1 67.92,64.8 v67.94,64.77
  Bottom 0.152: v8.89,3.81 v15.24,3.81 31.11,3.81 33.02,1.91 69.22,1.91 71.91,4.6 71.91,6.19 76.2,10.48 77.79,10.48 94.93,27.62 v94.93,27.94 94.85,27.86 93.74,27.86 84.14,37.47 84.14,45.4 v83.82,45.72 | v77.44,61.79 77.44,51.46 78.74,50.16 v78.74,49.21
ALU/IN/Z2/N3  (via drill 0.35)
  Top 0.152: v27.94,8.89 IC14.9 | IC70.4 96.52,20.95 95.57,21.91 95.57,23.08 95.25,23.39 IC70.12 v95.25,26.67 | IC30.2 IC30.13 78.74,60.33 78.9,60.48 80.19,60.48 80.69,60.98 83.16,60.98 83.82,60.33 IC30.9 v83.82,57.15 IC30.6 | v121.92,68.58 IC52.1 | IC26.3 v64.14,71.75 | v14.08,13.22 13.97,13.11 IC15.9
  Route2 0.152: v64.14,71.75 65.41,73.03 66.36,73.03 76.2,63.18 80.01,63.18 83.82,59.37 v83.82,57.15 88.65,57.15 91.06,59.56 114.17,59.56 121.92,67.31 v121.92,68.58
  Route3 0.152: v14.08,13.22 23.61,13.22 v27.94,8.89 28.57,8.26 v28.57,2.54
  Bottom 0.152: v83.82,57.15 85.09,57.15 89.72,52.52 89.72,51.16 89.53,50.98 89.53,48.51 88.65,47.62 88.65,45.85 89.53,44.96 89.53,34.92 91.47,32.99 91.47,31.5 93.09,29.87 94.59,29.87 95.73,28.73 95.73,27.15 v95.25,26.67 78.26,9.68 76.36,9.68 72.71,6.03 72.71,4.13 69.85,1.27 33.02,1.27 31.75,2.54 v28.57,2.54
ALU/OUT/N0  (via drill 0.35)
  Top 0.152: IC7.6 113.67,82.65 115.67,80.64 v117.89,80.64 118.11,80.64 120.02,78.74 121.92,78.74 IC53.1 | IC2.3 v109.86,74.52
  Route15 0.152: v109.86,74.52 109.86,75.63 114.87,80.64 v117.89,80.64
ALU/OUT/N1  (via drill 0.35)
  Top 0.152: IC2.5 112.39,74.45 112.87,74.93 112.87,77.31 v113.19,77.63 | IC7.10 114.94,89.09 v115,89.03 | IC53.13 123.19,86.36 122.56,87 v117.47,87
  Bottom 0.152: v115,89.03 115,89 117,87 v117.47,87 117.47,81.28 113.82,77.63 v113.19,77.63
ALU/OUT/N2  (via drill 0.35)
  Top 0.152: v98.42,57.15 IC5.6 | v92.71,74.93 IC54.1 | v114.88,71.66 114.94,71.72 IC2.7
  Route14 0.152: v92.71,74.93 94.93,74.93 98.42,71.44 109.57,71.44 v109.73,71.28 110.08,71.63 114.85,71.63 v114.88,71.66
  Bottom 0.152: v98.42,57.15 98.42,57.66 108.08,67.31 108.08,69.63 v109.73,71.28
ALU/OUT/N3  (via drill 0.35)
  Top 0.152: v116.2,76.2 IC2.9 | IC5.10 99.69,60.42 v99.67,60.45 | v99.54,76.2 97.47,76.2 97.44,76.23 95.67,76.23 93.98,77.92 IC54.13
  Route2 0.152: v100.97,66.04 100.57,65.64 100.57,61.35 v99.67,60.45
  Route3 0.152: v99.54,76.2 100.33,76.2 101.28,75.25 110.81,75.25 111.76,76.2 113.35,76.2 113.98,76.84 115.57,76.84 v116.2,76.2
  Bottom 0.152: v99.54,76.2 99.54,73.34 98.42,72.23 98.42,68.58 v100.97,66.04
ASH  (via drill 0.35)
  Top 0.152: v114.46,54.61 114.46,52.97 IC68.6 | v121.28,54.61 121.92,54.61 123.19,53.34 IC61.13 | IC6.2 IC6.13 78.74,92.08 79.38,92.71 83.19,92.71 83.82,92.08 IC6.9 IC6.6 83.82,83.19 84.45,82.55 v84.45,81.92
  Route14 0.152: v114.46,54.61 109.86,54.61 84.45,80.01 v84.45,81.92
  Route15 0.152: v114.46,54.61 115.09,53.98 120.65,53.98 v121.28,54.61
B/IN/N0  (via drill 0.35)
  Top 0.152: v144.78,38.73 IC55.9 | v144.78,67.63 IC58.9 | v144.78,77.79 IC59.9 | IC60.9 144.78,88.9 v145.41,88.27 | v128.27,53.98 IC61.9 128.27,51.12 128.91,50.48 v128.91,49.21 | v128.91,60.01 128.27,60.64 IC62.9 | IC64.3 124.46,22.86 v126.36,20.95 | v144.78,21.59 145.1,21.59 145.41,21.27 IC4.7 | v144.78,47.31 IC56.9 | IC57.9 144.78,57.68 145.31,57.15 v145.41,57.15
  Route2 0.152: v128.91,60.01 129.54,59.37 129.54,55.25 v128.27,53.98
  Route3 0.152: v126.36,20.95 128.91,23.49 128.91,29.05 130.97,31.11 130.97,36.2 128.27,38.89 128.27,42.86 129.86,44.45 129.86,48.26 v128.91,49.21 | v145.41,88.27 145.41,78.42 v144.78,77.79 146.53,76.04 146.53,69.37 v144.78,67.63 144.15,66.99 144.15,65.25 144.78,64.61 144.78,57.79 v145.41,57.15 145.41,47.94 v144.78,47.31 144.62,47.15 144.62,38.89 v144.78,38.73
  Bottom 0.152: v126.36,20.95 144.15,20.95 v144.78,21.59 147.32,24.13 147.32,36.2 v144.78,38.73
B/IN/N1  (via drill 0.35)
  Top 0.152: v140.97,61.59 IC58.3 | v144.15,50.48 143.51,49.85 IC56.10 | v126.84,26.51 125.73,25.4 IC64.4 | v139.7,39.37 140.97,40.64 IC56.3 | v124.46,54.61 IC62.3 | IC62.10 127,59.69 v128.27,58.42 | IC4.9 146.69,31.75 147.96,33.02 147.96,81.92 v147.32,82.55 147.32,92.08 146.69,92.71 144.15,92.71 143.51,92.08 IC60.10 | IC60.3 v140.97,82.55 | IC58.10 143.51,67.63 v145.41,65.72
  Route2 0.152: v124.46,54.61 v128.27,58.42 | v140.97,82.55 v147.32,82.55
  Route3 0.152: v139.7,39.37 v124.46,54.61
  Route15 0.152: v145.41,65.72 141.29,61.59 v140.97,61.59 140.97,60.58 143.19,58.36 143.19,53.34 144.15,52.39 v144.15,50.48 146.05,48.58 146.05,47.08 139.7,40.73 v139.7,39.37
  Bottom 0.152: v126.84,26.51 127.64,26.51 139.7,38.58 v139.7,39.37 | v140.97,82.55 137.32,78.9 137.32,77.63 130.25,70.56 130.25,59.77 128.91,58.42 v128.27,58.42
B/IN/N2  (via drill 0.35)
  Top 0.152: IC61.11 v125.73,54.61 IC62.4 IC62.11 | IC64.10 127,31.75 v128.27,33.02 | IC61.4 v125.73,44.45 | IC58.4 142.24,61.7 142.88,61.06 v142.88,60.96 142.88,60.86 142.24,60.22 IC57.11 v142.24,57.15 | v144.15,29.21 IC4.11 | IC57.4 v142.24,51.44 | IC58.11 v142.24,67.63
  Route2 0.152: v144.15,29.21 144.15,35.72 146.39,37.96 146.39,48.08 145.18,49.29 144.38,49.29 v142.24,51.44 | v142.24,67.63 143.35,66.52 143.35,61.44 v142.88,60.96
  Route3 0.152: v142.24,51.44 140.97,51.44 138.59,53.82 135.25,53.82 133.67,52.23 128.11,52.23 v125.73,54.61
  Route15 0.152: v128.27,33.02 129.54,33.02 130.49,33.97 130.49,38.64 128.27,40.86 128.27,41.91 v125.73,44.45 125.75,44.47 v125.75,50.96
  Bottom 0.152: v125.73,54.61 125.73,51.28 125.75,51.25 v125.75,50.96 | v142.24,51.44 v142.24,57.15
B/IN/N3  (via drill 0.35)
  Top 0.152: v140.97,77.79 IC59.12 | IC60.12 140.97,88.9 143.51,86.36 IC60.5 143.51,81.92 v142.88,81.28 | v127,55.25 IC62.5 | v127.64,29.21 127,29.21 125.73,30.48 IC64.11 | IC4.14 v140.34,24.13 | v128.27,44.45 127,45.72 IC61.5 127,47.62 124.46,50.16 IC61.12 124.49,52.58 v124.49,51.42 | IC62.12 124.46,60.96 v122.56,59.05 | IC59.5 v143.51,71.75
  Route2 0.152: v127.64,29.21 135.25,29.21 v140.34,24.13 | v140.97,77.79 140.97,79.38 v142.88,81.28 142.88,72.39 v143.51,71.75 140.95,69.19 140.95,66.08 142.24,64.79 v142.24,64.77
  Route14 0.152: v128.27,44.45 138.43,44.45 141.29,47.31 141.29,57.47 143.83,60.01 143.83,63.18 v142.24,64.77 | v127,55.25 127,53.93 v124.49,51.42
  Route15 0.152: v122.56,59.05 123.19,59.05 v127,55.25
  Bottom 0.152: v128.27,44.45 128.27,40.64 131.29,37.62 131.29,32.86 v127.64,29.21
C/ADD  (via drill 0.35)
  Top 0.152: IC49.1 48.1,73.28 48.1,75.41 48.9,76.2 50.8,76.2 | 53.34,76.2 50.8,76.2 | 50.8,76.2 IC49.12 | 53.34,76.2 IC49.5 | v93.98,39.37 IC10.13 | v111.76,57.15 112.39,57.15 113.03,57.79 IC68.10 113.03,60.01 v113.67,60.64 | v115.57,65.88 IC69.8 | 55.88,78.74 58.42,78.74 v59.69,77.47 | 55.88,78.74 IC49.8 | 55.88,78.74 55.88,77.15 54.93,76.2 53.34,76.2
  Route2 0.152: v111.76,57.15 95.89,41.28 | 95.89,41.28 v93.98,39.37 | v59.69,77.47 62.23,74.93 62.23,72.39 64.61,70.01 66.52,70.01 78.11,58.42 78.11,56.31 79.17,55.25 81.92,55.25 95.89,41.28
  Route15 0.152: v115.57,65.88 115.57,64.93 113.67,63.02 113.67,62.55 113.03,61.91 113.03,61.28 v113.67,60.64
C/MU1  (via drill 0.35)
  Top 0.152: IC69.12 v110.49,64.45 IC69.3 | IC50.1 48.26,86.36 48.9,87 49.53,87 50.8,88.27 50.8,88.9 | 50.8,88.9 IC50.12 50.8,93.03 51.44,93.66 54.93,93.66 55.88,92.71 IC50.8 55.88,90.81 57.15,90.81 v58.42,89.53 | IC50.5 53.34,86.36 50.8,88.9
  Route15 0.152: v110.49,64.45 109.54,64.45 105.41,68.58 91.6,68.58 90.96,67.95 84.93,67.95 84.3,68.58 79.38,68.58 68.58,79.38 66.36,79.38 65.41,80.33 65.41,82.55 v58.42,89.53
C/MU2  (via drill 0.35)
  Top 0.152: IC51.1 92.71,65.09 95.25,67.63 IC51.12 95.25,69.85 97.16,71.75 100.97,71.75 v101.6,72.39 | IC51.5 97.79,65.41 v99.06,66.67 | IC51.8 100.33,69.85 v101.6,69.85 | v109.08,67.59 109.22,67.73 IC69.13 | v111.67,61.59 111.67,62.88 IC69.4
  Route3 0.152: v99.06,66.67 101.6,69.22 v101.6,69.85
  Route15 0.152: v104.78,70.48 107.67,67.59 v109.08,67.59 109.72,67.59 110.63,66.67 111.76,66.67 113.03,65.41 113.03,62.96 v111.67,61.59
  Bottom 0.152: v101.6,69.85 101.6,70.48 | 101.6,70.48 v101.6,72.39 | 101.6,70.48 v104.78,70.48
C/SUB  (via drill 0.35)
  Top 0.152: IC69.9 v114.3,67.63 | IC48.1 7.62,72.39 8.26,71.75 12.06,71.75 12.7,72.39 IC48.5 12.7,74.8 10.16,77.34 IC48.12 10.16,80.64 10.79,81.28 14.61,81.28 15.24,80.64 IC48.8 15.34,79.38 v20.95,79.38 | v111.73,60.52 111.73,58.98 IC68.11
  Route14 0.152: v114.3,67.63 114.36,67.63 114.81,67.18 116.17,67.18 116.36,66.99 116.36,63.98 115.13,62.74 113.95,62.74 v111.73,60.52
  Route15 0.152: v20.95,79.38 41.27,59.05 56.83,59.05 59.05,61.28 60.8,61.28 63.02,59.05 110.27,59.05 v111.73,60.52
CCF  (via drill 0.35)
  Top 0.152: v121.92,48.26 IC61.1 | IC47.12 v97.16,92.71
  Route2 0.152: v97.16,92.71 118.75,92.71 130.18,81.28 130.18,64.77 120.17,54.77 120.17,50.01 v121.92,48.26
CLK  (via drill 0.35)
  Top 0.152: IC47.13 95.89,88.58 94.61,87.31 IC47.3 v94.61,82.55 | v93.03,27.62 92.71,27.94 IC10.1 v92.71,31.43 94.3,31.43 95.73,32.86 96.84,32.86 97.79,31.91 IC10.5
  Route15 0.152: v93.03,27.62 111.76,8.89 RCLK.1
  Bottom 0.152: RCLK.1 113.03,5.08 118.11,5.08 CLK.1 | v94.61,82.55 94.46,82.39 94.46,75.25 93.31,74.1 93.31,63.28 94.23,62.36 94.23,56.77 93.34,55.88 93.34,49.69 91.92,48.26 91.92,45.24 92.71,44.45 92.71,39.21 94.14,37.78 94.14,36.83 92.71,35.4 v92.71,31.43
CMPA/OUT  (via drill 0.35)
  Top 0.152: IC10.8 100.33,37.47 102.55,39.69 v102.55,65.09 | v100.33,81.28 100.33,81.92 99.69,82.55 IC47.7 | v66.67,80.64 IC26.12
  Route3 0.152: v100.33,81.28 99.22,80.17 91.92,80.17 91.44,80.64 81.12,80.64 80.33,79.85 76.36,79.85 75.56,80.64 v66.67,80.64
  Bottom 0.152: v102.55,65.09 102.55,67.37 100.33,69.6 v100.33,81.28
CSF  (via drill 0.35)
  Top 0.152: IC47.4 95.89,85.73 v96.52,86.36 | v122.56,60.33 123.19,60.96 IC62.13
  Route15 0.152: v122.56,60.33 110.49,72.39 108.58,72.39 104.14,76.84 104.14,78.74 v96.52,86.36
GND  (via drill 0.35)
  Top 0.152: v146.69,21.27 IC4.8 | 146.69,41.91 147.32,41.28 147.32,35.24 146.05,33.97 v146.05,33.66 IC55.7 | 146.69,41.91 146.05,42.55 IC56.7 | 146.69,41.91 146.69,50.16 146.05,50.8 IC57.7 146.05,54.61 146.69,55.25 146.69,60.96 146.05,61.59 IC58.7 146.05,64.45 146.69,65.09 146.69,71.12 146.05,71.75 IC59.7 146.05,74.61 146.69,75.25 146.69,80.64 146.05,81.28 IC60.7 | IC66.7 115.57,34.29 116.2,34.92 116.2,40.64 115.57,41.28 IC67.7 115.57,42.7 116.52,42.7 117.63,43.82 117.63,49.21 116.84,50.01 116.84,51.12 116.68,51.28 115.73,51.28 115.57,51.44 IC68.7 115.79,53.02 116.84,53.02 118.75,54.93 118.75,58.42 115.57,61.59 IC69.7 115.57,64.77 116.82,66.02 116.82,69.83 v116.84,69.85 116.84,71.28 116.2,71.91 IC2.8 | IC52.7 129.54,64.77 130.18,64.14 130.18,58.74 129.54,58.1 IC62.7 129.54,54.61 130.49,53.66 130.49,49.21 129.54,48.26 IC61.7 129.54,45.09 130.33,44.29 130.33,38.26 129.54,37.47 IC63.7 v129.54,34.29 | 69.85,52.71 68.58,52.71 IC17.6 | IC22.6 68.58,62.87 69.85,62.87 IC22.7 71.12,64.24 71.12,71.12 70.48,71.75 IC26.8 | IC22.9 68.58,67.69 69.22,67.05 69.22,64.87 68.58,64.24 IC22.6 | IC42.6 68.58,41.28 69.85,41.28 IC42.7 | 69.85,18.41 68.58,18.41 IC32.6 | 69.85,29.84 68.58,29.84 IC37.6 | 69.85,29.84 69.85,28.26 70.8,27.3 70.8,20.64 69.85,19.68 IC32.7 69.85,18.41 | 69.85,29.84 IC37.7 69.85,32.07 71.75,33.97 71.75,38.1 69.85,40.01 IC42.7 | 69.85,52.71 69.85,50.96 70.48,50.32 70.48,42.55 69.85,41.91 IC42.7 | 69.85,52.71 IC17.7 | IC65.7 115.57,7.62 GND.1 | IC64.7 v129.54,22.86 130.49,21.91 130.49,9.84 128.27,7.62 128.27,5.71 127.64,5.08 118.11,5.08 GND.1
  Top 0.152: IC28.7 85.09,28.57 86.36,27.3 86.36,21.27 85.09,20 IC27.7 85.09,17.14 81.92,13.97 v74.3,13.97 | IC14.7 29.21,5.71 31.75,5.71 36.2,1.27 65.41,1.27 68.63,4.5 68.63,5.77 | IC11.7 69.85,5.71 68.68,5.71 68.63,5.77 | IC11.7 69.85,9.53 v74.3,13.97 | GND.1 114.94,4.45 69.85,4.45 IC11.7 | v74.3,13.97 72.39,13.97 69.85,16.51 69.85,18.41 | IC70.7 100.33,20.42 101.6,21.69 101.6,27.41 100.33,28.68 IC10.7 v100.33,31.75 | IC5.12 97.16,54.61 95.89,53.34 IC5.4 v95.89,50.8 95.89,49.53 97.16,48.26 IC3.12 97.16,45.09 96.52,44.45 | IC3.4 95.89,43.82 96.52,44.45 | IC3.8 100.97,41.28 99.69,41.28 IC3.7 | 100.97,52.71 99.69,52.71 IC5.7 | 100.97,52.71 IC3.9 100.97,46.36 | 100.97,52.71 IC5.8 IC5.9 100.97,60.33 100.33,60.96 IC51.7 | IC47.11 98.42,90.81 99.69,90.81 IC47.10 99.69,92.33 101.35,93.98 110.36,93.98 112.39,91.95 | IC47.11 98.42,86.36 | 98.42,86.36 IC47.6 IC47.5 97.16,82.87 96.84,82.55 v95.89,82.55 | IC54.7 100.33,74.93 101.44,76.04 101.44,84.08 IC47.8 100.97,86.04 100.65,86.36 98.42,86.36 | IC7.7 114.94,84.45 116.2,84.45 IC7.8 | IC7.8 IC7.9 116.2,92.46 115.82,92.84 113.28,92.84 112.39,91.95 | IC53.7 129.54,76.84 127.79,75.09 v124.78,75.09 | 112.39,91.95 IC7.12 112.39,89.15 111.12,87.88 IC7.4 v111.12,83.03 | 84.45,73.03 85.72,73.03 IC1.8 85.72,74.24 86.52,75.03 86.52,77.21 85.72,78 IC1.9 85.72,82.17 85.09,82.8 IC6.7 85.09,85.09 90.93,90.93 90.93,92.58 92.33,93.98 97.66,93.98 98.42,93.22 IC47.11 | IC1.12 81.92,77.79 80.64,76.52 IC1.4 v80.64,71.75 | v84.45,71.75 84.45,73.03 | 84.45,73.03 IC1.7 | v84.45,50.8 84.77,50.8 85.09,51.12 IC30.7 | 15.24,66.67 v15.24,66.04 IC25.7 | 15.24,66.67 13.97,67.95 IC25.9 13.97,69.85 15.24,71.12 IC48.7
  Top 0.152: IC19.11 24.13,57.79 v24.61,57.31 24.77,57.15 v27.94,57.15 IC19.7 27.94,51.75 31.75,47.94 31.75,45.5 29.21,42.96 IC44.7 29.21,38.1 30.8,36.51 30.8,32.51 | 24.13,71.12 26.04,71.12 26.67,70.48 IC24.9 26.67,67.31 27.94,66.04 IC24.7 v27.94,61.59 | 15.24,66.67 19.68,71.12 24.13,71.12 | 24.13,71.12 IC24.11 | IC34.7 29.21,20.64 30.72,22.15 30.72,25.32 29.21,26.83 IC39.7 29.21,31.43 30.29,32.51 30.8,32.51 | v21.59,64.45 IC24.2 | v16.19,53.34 15.24,53.34 IC20.7 | v8.89,64.77 IC25.2 | v15.24,39.37 IC45.7 | v16.51,6.35 15.24,6.35 IC15.7 | v57.15,84.45 55.88,84.45 IC50.7 | v64.14,80.96 IC26.14 | v68.58,82.55 IC9.7 | IC49.7 55.88,71.75 54.61,70.48 IC21.9 54.61,68 55.09,67.53 55.09,64.71 54.61,64.24 IC21.6 54.61,62.87 55.88,62.87 IC21.7 55.88,61.91 56.04,61.75 60.8,61.75 61.28,61.28 61.28,59.21 55.88,53.82 IC16.7 55.88,52.71 | IC41.6 55.88,41.28 57.15,41.28 IC41.7 57.15,42.55 | 55.88,52.71 54.61,52.71 IC16.6 | 57.15,42.55 57.15,43.18 59.37,45.4 59.37,48.26 55.88,51.75 55.88,52.71 | v43.18,53.34 41.91,53.34 IC18.7 | v44.45,30.48 43.18,30.48 IC38.7 | v45.72,43.82 45.72,43.02 44.08,41.38 IC43.7 | v58.42,42.55 57.15,42.55 | 57.15,29.84 55.88,29.84 IC36.6 | 56.52,18.41 57.15,18.41 IC31.7 | 56.52,18.41 55.88,18.41 IC31.6 | 55.88,6.03 IC12.7 | 56.52,18.41 v56.52,15.24 56.83,14.92 56.83,6.35 56.52,6.03 55.88,6.03 | 57.15,29.84 IC36.7 | v41.91,64.45 IC23.7 | v44.45,19.05 43.18,19.05 IC33.7 | v33.91,32.51 30.8,32.51 | IC3.8 v100.97,40.01 | v57.15,28.6 57.15,29.84 | 55.88,6.03 54.83,6.03 IC12.6 54.61,6.98 53.82,7.78 45.14,7.78 IC13.7 | IC22.6 68.58,61.7 68.2,61.31 v65.38,61.31 | IC11.6 68.63,5.77 | IC8.7 v85.09,61.59
  Top 0.152: IC29.7 85.09,39.69 83.82,38.42 82.39,38.42 81.76,39.05 v80.64,39.05 | IC7.8 120.12,80.64 v120.97,80.64 | IC40.7 v15.24,28.42 16.35,27.3 16.35,18.99 15.88,18.52 IC35.7 | IC3.8 100.97,42.55 101.6,43.18 101.6,45.72 100.97,46.36 | 96.52,44.45 99.38,44.45 100.97,46.04 100.97,46.36
  Route2 0.152: v146.05,33.66 146.69,33.02 146.69,24.29 | 146.69,24.29 v146.69,21.27 | 146.69,24.29 v141.6,24.29
  Route3 0.152: v8.89,64.77 10.16,66.04 v15.24,66.04 | v100.97,40.01 100.97,32.38 v100.33,31.75 | v84.45,50.8 85.09,51.44 85.09,51.59 86.84,53.34 86.84,59.85 v85.09,61.59
  Route15 0.152: v50.48,22.54 56.54,28.6 v57.15,28.6 | v124.94,37.94 124.94,39.55 123.8,40.69 123.8,44.63 v123.67,44.77
  Bottom 0.152: 141.6,76.2 141.6,74.93 140.34,73.66 140.34,67.95 141.6,66.67 141.6,66.04 C40.2 141.29,63.82 140.18,62.7 140.18,59.53 141.29,58.42 C38.2 C37.2 141.6,45.72 141.6,42.7 140.81,41.91 140.81,40.16 141.6,39.37 141.6,34.29 C35.2 141.29,29.52 141.6,29.21 v141.6,24.29 141.6,22.86 C34.2 140.34,22.86 138.75,24.45 137.32,24.45 135.73,22.86 v129.54,22.86 128.91,22.86 125.09,26.67 125.09,27.94 124.94,27.94 | 141.6,76.2 141.6,77.15 142.24,77.79 142.24,80.01 141.6,80.64 141.6,81.6 142.56,82.55 142.56,84.45 141.13,85.88 141.13,87.47 C61.2 | 141.6,76.2 C5.2 | 124.94,33.97 v124.94,37.94 124.94,39.37 C57.2 | 124.94,33.97 124.94,27.94 | 125.09,59.69 125.09,63.34 125.57,63.82 125.57,68.26 125.09,68.74 125.09,69.85 C6.2 124.78,70.17 | 125.09,59.69 C59.2 | 124.78,70.17 v124.78,75.09 C41.2 124.14,80.64 v120.97,80.64 | v123.67,44.77 122.87,45.56 122.87,47.62 C58.2 123.51,50.8 123.51,54.04 123.8,54.34 123.8,54.88 125.09,56.18 125.09,59.69 | v116.84,69.85 122.24,69.85 122.87,70.48 124.46,70.48 124.78,70.17 | 124.94,27.94 C56.2 | C22.2 95.57,82.87 v95.89,82.55 96.52,81.92 96.52,80.8 95.57,79.85 C15.2 95.57,73.98 96.04,73.5 96.04,69.53 95.89,69.37 95.89,66.04 C10.2 95.57,63.97 96.52,63.02 96.52,57.79 95.89,57.15 95.89,55.88 | C54.2 95.89,21.59 95.89,25.56 97.18,26.85 97.18,28.55 95.57,30.16 C3.2 95.89,33.02 95.89,44.45 C66.2 93.98,46.04 93.98,48.26 95.89,50.16 v95.89,50.8 95.89,55.88 | 95.89,55.88 C39.2 | C11.2 111.12,22.86 111.12,34.29 C1.2 110.49,34.29 110.49,36.2 107.95,38.73 107.95,40.01 108.9,40.96 108.9,42.86 107.95,43.82 107.95,44.45 109.22,45.72 C36.2 110.65,45.88 110.65,48.1 109.54,49.21 109.54,51.28 111.12,52.86 111.12,55.88
  Bottom 0.152: C42.2 111.12,87.63 v111.12,83.03 110.81,82.71 110.81,75.88 | C7.2 111.12,76.2 110.81,75.88 | 111.12,55.88 111.12,56.04 110.65,56.52 110.65,59.53 110.17,60.01 109.22,60.01 108.58,60.64 108.58,64.45 110.17,66.04 C60.2 110.81,75.88 | 111.12,55.88 C4.2 | 80.64,76.2 v80.64,71.75 | 80.64,76.2 80.64,78.9 79.06,80.49 79.06,82.55 80.64,84.14 80.64,87.63 C21.2 | 80.64,76.2 C16.2 | 80.49,66.04 80.64,66.04 80.64,64.45 78.74,62.55 78.74,56.52 79.38,55.88 C63.2 80.64,55.88 80.64,54.93 84.45,51.12 v84.45,50.8 84.45,50.32 80.64,46.51 80.64,44.45 C65.2 80.33,39.37 v80.64,39.05 80.64,33.02 C2.2 80.33,30 81.28,29.05 81.28,27.62 80.64,26.99 80.64,21.59 C55.2 80.33,20 v74.3,13.97 67.94,7.62 66.04,7.62 64.77,8.89 C71.2 65.09,15.24 | 80.49,66.04 C12.2 | 23.5,57.31 23.5,55.88 C8.2 22.86,55.88 | v21.59,64.45 C29.2 23.5,66.04 23.5,62.87 22.86,62.23 22.86,57.94 23.5,57.31 | C24.2 C31.2 10.16,55.88 12.7,53.34 v16.19,53.34 16.99,54.13 21.11,54.13 22.86,55.88 | C24.2 10.48,66.67 10.95,67.15 10.95,75.73 C23.2 | v8.89,64.77 10.16,66.04 C24.2 | C67.2 10.79,8.89 10.79,11.11 7.78,14.13 7.78,20.16 9.21,21.59 C72.2 10.79,21.59 10.79,23.34 8.73,25.4 8.73,26.51 9.84,27.62 14.45,27.62 v15.24,28.42 | 24.77,33.02 24.77,36.07 25.65,36.96 25.65,38.73 24.92,39.47 24.92,44.45 C45.2 24.13,44.45 24.13,54.61 22.86,55.88 | 24.77,14.61 24.77,8.89 C68.2 | 24.77,14.61 26.35,16.19 26.35,19.37 24.13,21.59 C52.2 24.77,21.59 24.77,24.13 24.45,24.45 24.45,26.35 25.08,26.99 25.08,27.94 24.77,28.26 24.77,33.02 | 24.77,14.61 v16.51,6.35 | 24.77,33.02 C32.2 24.29,32.86 19.68,32.86 v15.24,28.42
